(* Logix 5000 AddOnInstructionDefinition export Banner_Q90RKU_Param_v4; software revision 33.00 *)

TYPE Banner_IOL_Port_v4 :   // UDT that has all of the data items necessary to communicate with a specific Port on a IO-Link Master
STRUCT
   Port_Controlled : INT;   // Each bit represents a port on an IO-Link Master. Set to 1 to tell AOI to control that port.
   Port_Activate : INT;   // Each bit represents a port on an IO-Link Master. When ON that port will process any commands in queue.
   Port_Read : INT;   // Each bit represents a port on an IO-Link Master. Used to determine when device AOI has requested a Read command.
   Port_Write : INT;   // Each bit represents a port on an IO-Link Master. Used to determine when device AOI has requested a Write command.
   Port_RW_Complete : INT;   // Each bit represents a port on an IO-Link Master. Tells device AOI that Read or Write request has been completed.
   Port_Device_Read : INT;
   Data_Transfer : SINT[190];   // Array to transfer data from IO-Master to device AOIs.
END_STRUCT
END_TYPE

TYPE Banner_Q90RKU_Analog_v4 :
STRUCT
   AO1_SP1 : DINT;
   AO1_SP2 : DINT;
   AO1_Output_Type : INT;   // 0 = 4-20 mA, 128 = 0-10V, 129 = .5-4.5V
   AO1_Slope : SINT;   // 0 = Positive, 1 = Negative
   AO1_Loss_of_Signal : SINT;   // 0 = Hold, 1 = Low, 2 = High
   AO1_Average : SINT;   // 0 = 1, 1 = 2, 2= 4, 3 = 8, 4 = 16, 5 = 32, 6 = 64, 7 = 128, 8 = 256, 9 = 512
END_STRUCT
END_TYPE

TYPE Banner_Q90RKU_BDC_v4 :
STRUCT
   SP1 : DINT;   // Switchpoint SP1 switch point in Switch or Window mode.
   SP2 : DINT;   // Switchpoint 2. SP2 switch point in Window mode only.
   SP_Logic : INT;   // 0 = Light Operate, 1 = Dark Operate
   Mode : SINT;   // 1 = Switch Mode/Single Mode, 2 = Window Mode
   Hysteresis : INT;
   Delay_On : DINT;   // 0 to 60000 ms
   Delay_Off : DINT;   // 0 to 60000 ms
   Teach_Offset : DINT;   // Offset applied to taught switch point during single point teach.
END_STRUCT
END_TYPE

TYPE Banner_Q90RKU_Config_v4 :
STRUCT
   Response_Speed : SINT;   // 0 = Fast, 1 = Medium, 2 = Slow
   Peak_Select_Mode : SINT;   // 0 = Strongest Peak, 1 = First Peak
   Output_Polarity : SINT;   // 0 = NPN, 1 = PNP
   Process_Data_Filter_Time : INT;
   Process_Data_Layout : SINT;   // 0 = Digital Measurement Sensor, 1 = Distance and Excess Gain, 2 = Distance and Excess Gain with Binary Data
   Remote_Input_Mode : SINT;   // 0 = Disabled, 1 = Teach
   LEDs_Disabled : SINT;   // 0 = Enabled, 1 = Disabled.
   Amplitude_Threshold : DINT;   // 100 to 10000.
   Limit_Filter_Enabled : SINT;   // 0 = Disabled, 1 = Enabled. Rate of change filter for the distance measurement.
   Limit_Filter_Positive_Hold_Time : DINT;   // 50 to 3600000. Hold time for when distance change exceeds configured window.
   Limit_Filter_Negative_Hold_Time : DINT;   // 50 to 3600000. Hold time for when distance change exceeds configured window.
   Limit_Filter_Positive_Distance : DINT;   // 0 to 1000. Window size for distance changes going away from sensor (set to 0 to disable)
   Limit_Filter_Negative_Distance : DINT;   // 0 to 1000. Window size for distance changes goin towards sensor (set to 0 to disable)
END_STRUCT
END_TYPE

TYPE Banner_Q90RKU_Direct_v4 :
STRUCT
   Master_Cycle_Time : INT;
   Min_Cycle_Time : INT;
   M_Sequence_Capability : INT;
   IO_Link_Version_ID : INT;
   Process_Data_Input_Length : INT;
   Process_Data_Output_Length : INT;
   Combined_Vendor_ID : DINT;   // IO-Link Vendor ID
   Vendor_ID1 : INT;
   Vendor_ID2 : INT;
   Combined_Device_ID : DINT;   // IO-Link Device ID
   Device_ID1 : INT;
   Device_ID2 : INT;
   Device_ID3 : INT;
END_STRUCT
END_TYPE

TYPE Banner_Q90RKU_RD_v4 :   // UDT that stores the Read Data for a Q90RKU.
STRUCT
   Direct : Banner_Q90RKU_Direct_v4;
   Serial_Number : STRING;
   Teach_State : SINT;
   SP1_TP1 : SINT;
   SP1_TP2 : SINT;
   SP2_TP1 : SINT;
   SP2_TP2 : SINT;
   Status : Banner_Q90RKU_Status_v4;
   All_Time_Run_Time : DINT;   // Read only counter that tracks the total time sensor has been running since manufacture. Value in Hours.
   MDC_Lower_Limit : DINT;
   MDC_Upper_Limit : DINT;
   MDC_Unit : INT;
   MDC_Scale : SINT;
END_STRUCT
END_TYPE

TYPE Banner_Q90RKU_Status_v4 :
STRUCT
   Distance_Meaurement : DINT;
   Excess_Gain : DINT;   // Amount of singla measured over the minimum threshold.
   Stability : SINT;
   Fault_Status : SINT;   // 0 = No Fault, 1 = Fault Present
   Analog_Output_Value : DINT;
   Temperature : DINT;
   Last_Taught_Temperature : DINT;   // Internal Temperature the last time device was taught.
END_STRUCT
END_TYPE

TYPE Banner_Q90RKU_v4 :   // All of the parameters for a Q90RKU.
STRUCT
   Initial_Global_Read : BOOL;   // Determines if all of the IO-Link data has been read into the PLC yet
   Command : INT;   // Value placed in here will activate a read or write to a specifc IO-Link Index
   Read : Banner_Q90RKU_RD_v4;   // Read Only Data
   Write : Banner_Q90RKU_WD_v4;   // Write Data
   Archive : Banner_Q90RKU_WD_v4;   // Archive Data
   Reset : BOOL;   // Resets AOI. This will force a complete parameter read of the sensor.
END_STRUCT
END_TYPE

TYPE Banner_Q90RKU_WD_v4 :   // UDT that stores the Write Data for a T30RKU.
STRUCT
   System_Command : INT;   // See IODD file for list of commands that can be activated via the System Command interface
   Teach_in_Channel : SINT;   // 0 = Default, 1 = BDC1, 192 = AO1
   BDC1 : Banner_Q90RKU_BDC_v4;
   Config : Banner_Q90RKU_Config_v4;
   Resettable_Run_Time : DINT;
   All_Time_Run_Time_Event_Time : DINT;
   Resettable_Run_Time_Event_Time : DINT;
   Analog : Banner_Q90RKU_Analog_v4;
   Active_Sensing_Range_Near : DINT;
   Active_Sensing_Range_Far : DINT;
END_STRUCT
END_TYPE

ADD_ON_INSTRUCTION Banner_Q90RKU_Param_v4   (* revision 4.1, vendor Banner Engineering *)
// AOI to read and write parameter data to an IO-Link Q90R Analog.
VAR_IN_OUT
   Q90RKU : Banner_Q90RKU_v4; {required}
   Port_Data : Banner_IOL_Port_v4; {required}
END_VAR
VAR_INPUT
   Port : DINT; {required}
END_VAR
VAR
   Local_Control : DINT; {access None}
   Global_Read_Command_Value : INT; {access None}
   Global_Write_Command_Value : INT; {access None}
   Command_Being_Processed : BOOL; {access None}
   Update_Archive : BOOL; {access None}
   Index_Write_Inprocess : DINT; {access None}
   Index_Write_Control : DINT; {access None}
   Inprocess_Index : DINT; {access None}
END_VAR

ROUTINE Logic   (* ladder *)
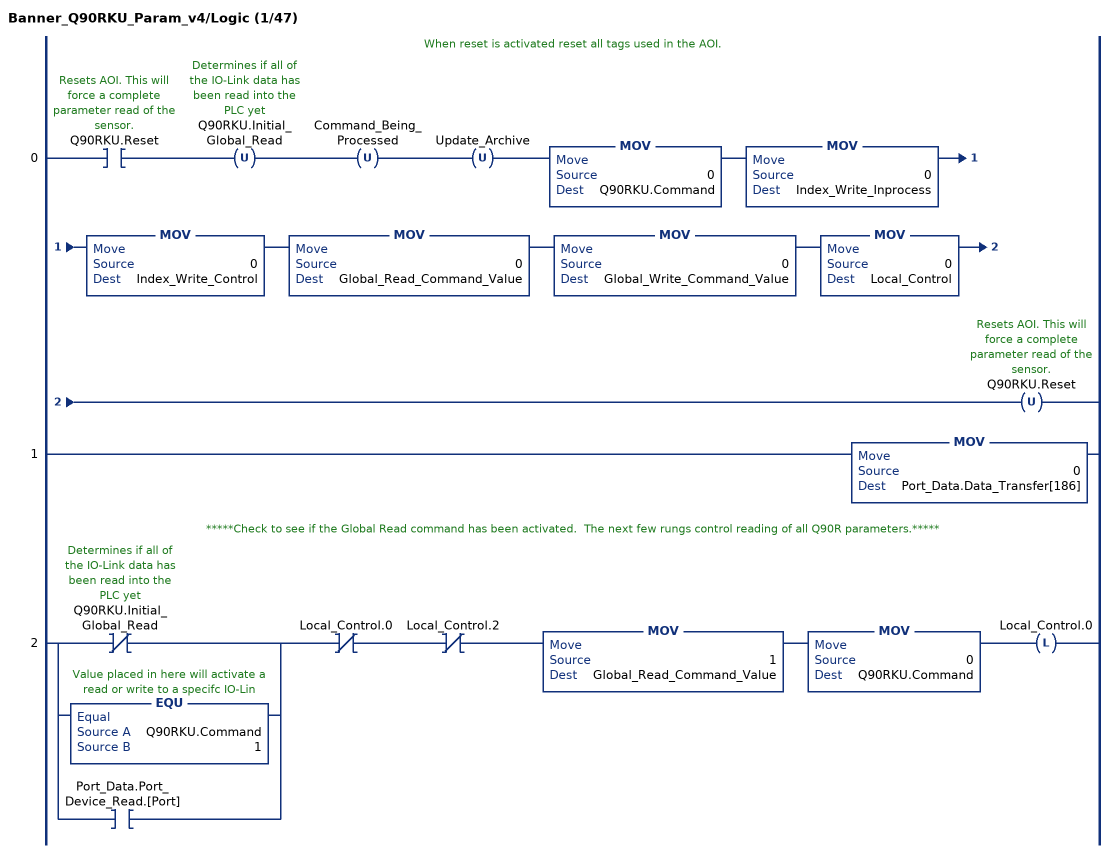
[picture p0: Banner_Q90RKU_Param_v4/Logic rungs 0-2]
   // When reset is activated reset all tags used in the AOI.
   0: XIC(Q90RKU.Reset)OTU(Q90RKU.Initial_Global_Read)OTU(Command_Being_Processed)OTU(Update_Archive)MOV(0,Q90RKU.Command)MOV(0,Index_Write_Inprocess)MOV(0,Index_Write_Control)MOV(0,Global_Read_Command_Value)MOV(0,Global_Write_Command_Value)MOV(0,Local_Control)OTU(Q90RKU.Reset);
   1: MOV(0,Port_Data.Data_Transfer[186]);
   // *****Check to see if the Global Read command has been activated.  The next few rungs control reading of all Q90R parameters.*****
   2: [XIO(Q90RKU.Initial_Global_Read) ,EQU(Q90RKU.Command,1) ,XIC(Port_Data.Port_Device_Read.[Port]) ]XIO(Local_Control.0)XIO(Local_Control.2)MOV(1,Global_Read_Command_Value)MOV(0,Q90RKU.Command)OTL(Local_Control.0);
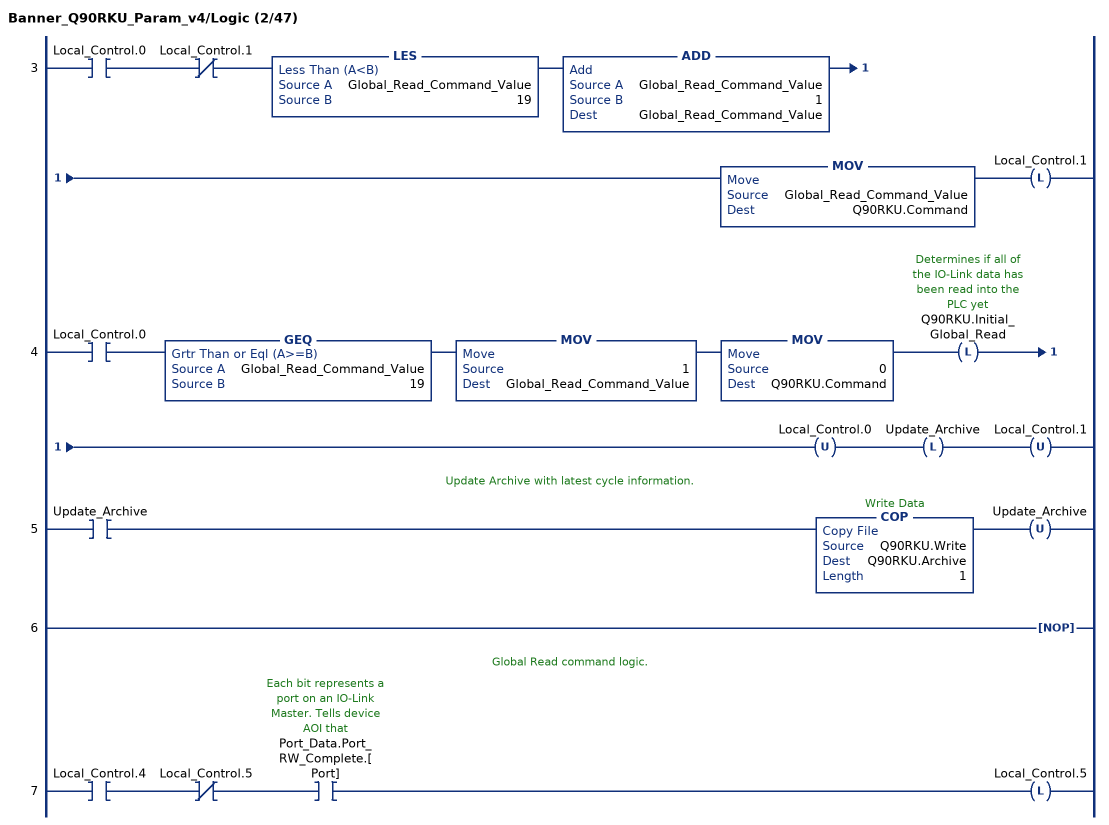
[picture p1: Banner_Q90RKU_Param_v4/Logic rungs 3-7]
   3: XIC(Local_Control.0)XIO(Local_Control.1)LES(Global_Read_Command_Value,19)ADD(Global_Read_Command_Value,1,Global_Read_Command_Value)MOV(Global_Read_Command_Value,Q90RKU.Command)OTL(Local_Control.1);
   4: XIC(Local_Control.0)GEQ(Global_Read_Command_Value,19)MOV(1,Global_Read_Command_Value)MOV(0,Q90RKU.Command)OTL(Q90RKU.Initial_Global_Read)OTU(Local_Control.0)OTL(Update_Archive)OTU(Local_Control.1);
   // Update Archive with latest cycle information.
   5: XIC(Update_Archive)COP(Q90RKU.Write,Q90RKU.Archive,1)OTU(Update_Archive);
   6: NOP();
   // Global Read command logic.
   7: XIC(Local_Control.4)XIO(Local_Control.5)XIC(Port_Data.Port_RW_Complete.[Port])OTL(Local_Control.5);
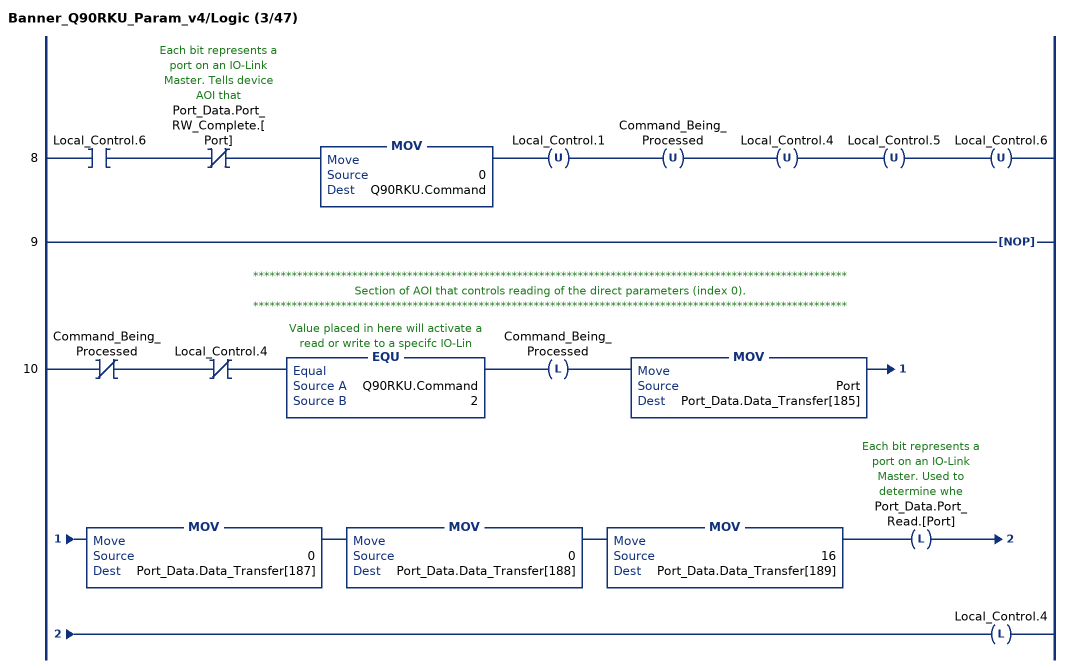
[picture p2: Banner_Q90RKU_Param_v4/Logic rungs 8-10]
   8: XIC(Local_Control.6)XIO(Port_Data.Port_RW_Complete.[Port])MOV(0,Q90RKU.Command)OTU(Local_Control.1)OTU(Command_Being_Processed)OTU(Local_Control.4)OTU(Local_Control.5)OTU(Local_Control.6);
   9: NOP();
   // ************************************************************************************************************
   // Section of AOI that controls reading of the direct parameters (index 0).
   // ************************************************************************************************************
   10: XIO(Command_Being_Processed)XIO(Local_Control.4)EQU(Q90RKU.Command,2)OTL(Command_Being_Processed)MOV(Port,Port_Data.Data_Transfer[185])MOV(0,Port_Data.Data_Transfer[187])MOV(0,Port_Data.Data_Transfer[188])MOV(16,Port_Data.Data_Transfer[189])OTL(Port_Data.Port_Read.[Port])OTL(Local_Control.4);
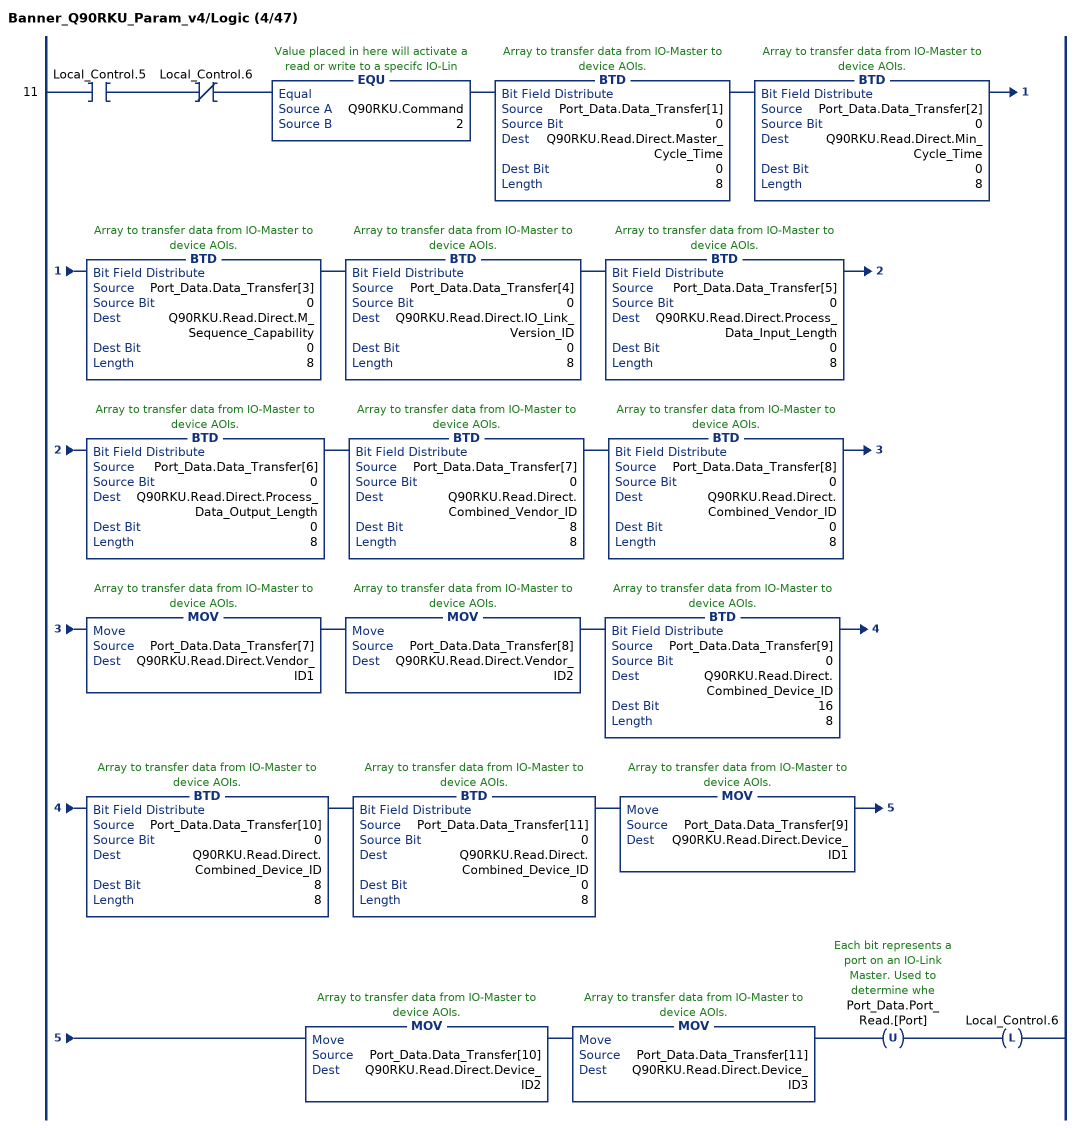
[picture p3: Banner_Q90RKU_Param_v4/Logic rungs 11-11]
   11: XIC(Local_Control.5)XIO(Local_Control.6)EQU(Q90RKU.Command,2)BTD(Port_Data.Data_Transfer[1],0,Q90RKU.Read.Direct.Master_Cycle_Time,0,8)BTD(Port_Data.Data_Transfer[2],0,Q90RKU.Read.Direct.Min_Cycle_Time,0,8)BTD(Port_Data.Data_Transfer[3],0,Q90RKU.Read.Direct.M_Sequence_Capability,0,8)BTD(Port_Data.Data_Transfer[4],0,Q90RKU.Read.Direct.IO_Link_Version_ID,0,8)BTD(Port_Data.Data_Transfer[5],0,Q90RKU.Read.Direct.Process_Data_Input_Length,0,8)BTD(Port_Data.Data_Transfer[6],0,Q90RKU.Read.Direct.Process_Data_Output_Length,0,8)BTD(Port_Data.Data_Transfer[7],0,Q90RKU.Read.Direct.Combined_Vendor_ID,8,8)BTD(Port_Data.Data_Transfer[8],0,Q90RKU.Read.Direct.Combined_Vendor_ID,0,8)MOV(Port_Data.Data_Transfer[7],Q90RKU.Read.Direct.Vendor_ID1)MOV(Port_Data.Data_Transfer[8],Q90RKU.Read.Direct.Vendor_ID2)BTD(Port_Data.Data_Transfer[9],0,Q90RKU.Read.Direct.Combined_Device_ID,16,8)BTD(Port_Data.Data_Transfer[10],0,Q90RKU.Read.Direct.Combined_Device_ID,8,8)BTD(Port_Data.Data_Transfer[11],0,Q90RKU.Read.Direct.Combined_Device_ID,0,8)MOV(Port_Data.Data_Transfer[9],Q90RKU.Read.Direct.Device_ID1)MOV(Port_Data.Data_Transfer[10],Q90RKU.Read.Direct.Device_ID2)MOV(Port_Data.Data_Transfer[11],Q90RKU.Read.Direct.Device_ID3)OTU(Port_Data.Port_Read.[Port])OTL(Local_Control.6);
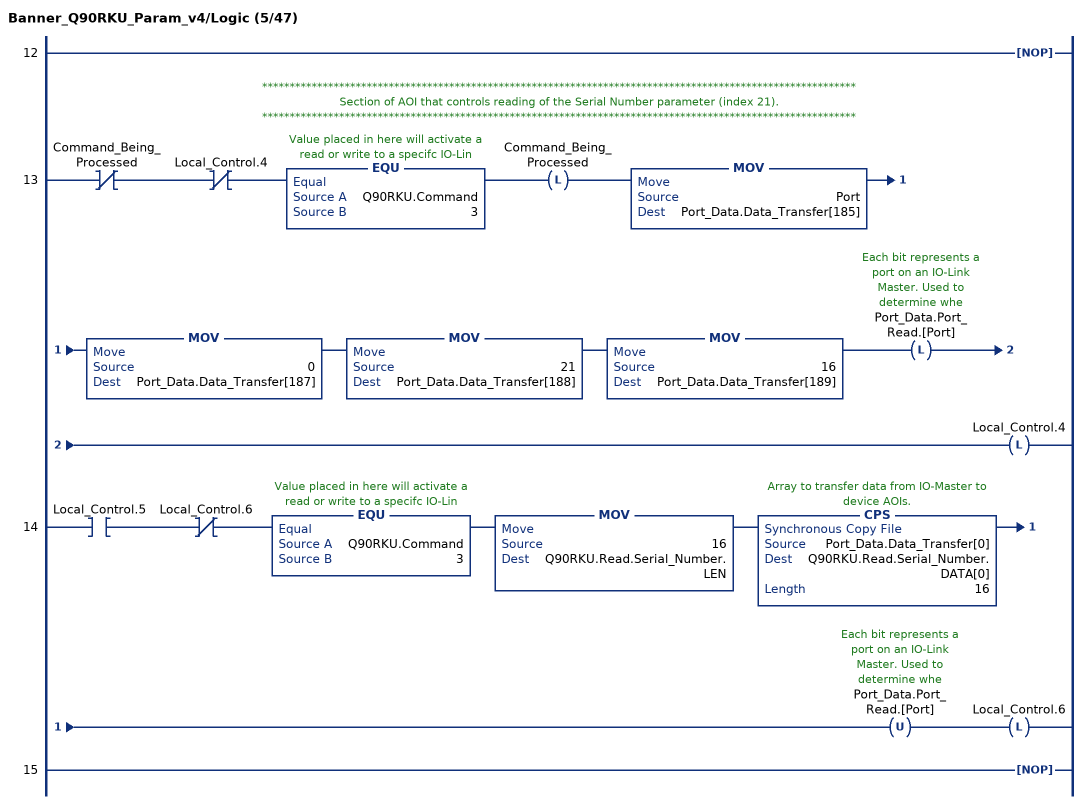
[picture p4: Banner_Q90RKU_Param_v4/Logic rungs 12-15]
   12: NOP();
   // ************************************************************************************************************
   // Section of AOI that controls reading of the Serial Number parameter (index 21).
   // ************************************************************************************************************
   13: XIO(Command_Being_Processed)XIO(Local_Control.4)EQU(Q90RKU.Command,3)OTL(Command_Being_Processed)MOV(Port,Port_Data.Data_Transfer[185])MOV(0,Port_Data.Data_Transfer[187])MOV(21,Port_Data.Data_Transfer[188])MOV(16,Port_Data.Data_Transfer[189])OTL(Port_Data.Port_Read.[Port])OTL(Local_Control.4);
   14: XIC(Local_Control.5)XIO(Local_Control.6)EQU(Q90RKU.Command,3)MOV(16,Q90RKU.Read.Serial_Number.LEN)CPS(Port_Data.Data_Transfer[0],Q90RKU.Read.Serial_Number.DATA[0],16)OTU(Port_Data.Port_Read.[Port])OTL(Local_Control.6);
   15: NOP();
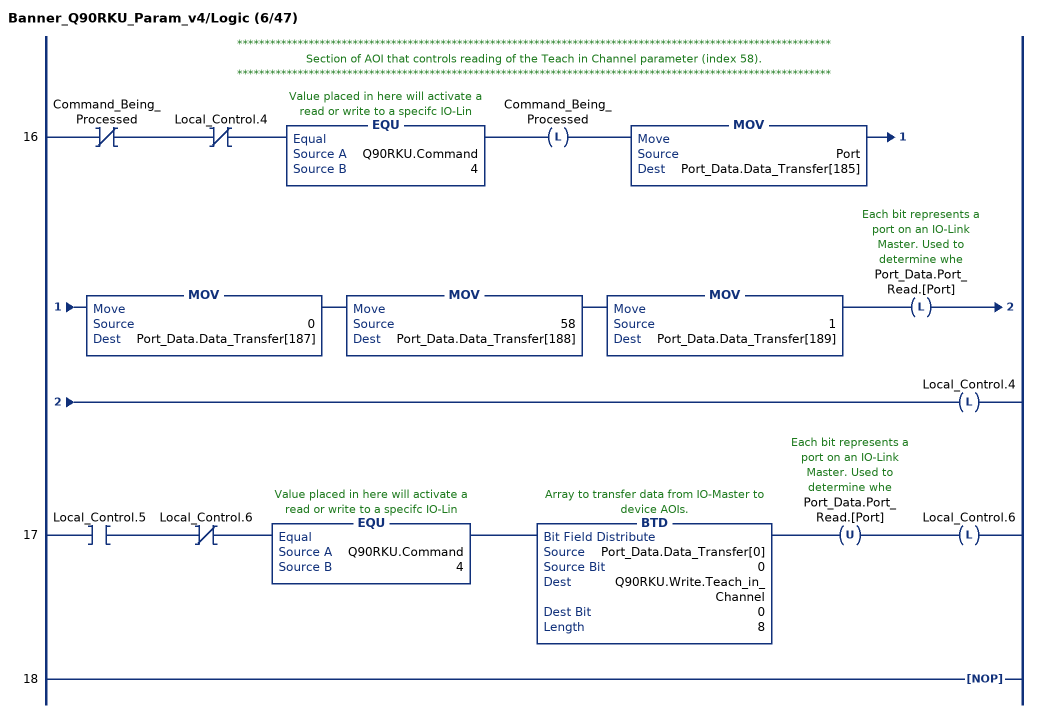
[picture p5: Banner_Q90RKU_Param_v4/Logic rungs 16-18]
   // ************************************************************************************************************
   // Section of AOI that controls reading of the Teach in Channel parameter (index 58).
   // ************************************************************************************************************
   16: XIO(Command_Being_Processed)XIO(Local_Control.4)EQU(Q90RKU.Command,4)OTL(Command_Being_Processed)MOV(Port,Port_Data.Data_Transfer[185])MOV(0,Port_Data.Data_Transfer[187])MOV(58,Port_Data.Data_Transfer[188])MOV(1,Port_Data.Data_Transfer[189])OTL(Port_Data.Port_Read.[Port])OTL(Local_Control.4);
   17: XIC(Local_Control.5)XIO(Local_Control.6)EQU(Q90RKU.Command,4)BTD(Port_Data.Data_Transfer[0],0,Q90RKU.Write.Teach_in_Channel,0,8)OTU(Port_Data.Port_Read.[Port])OTL(Local_Control.6);
   18: NOP();
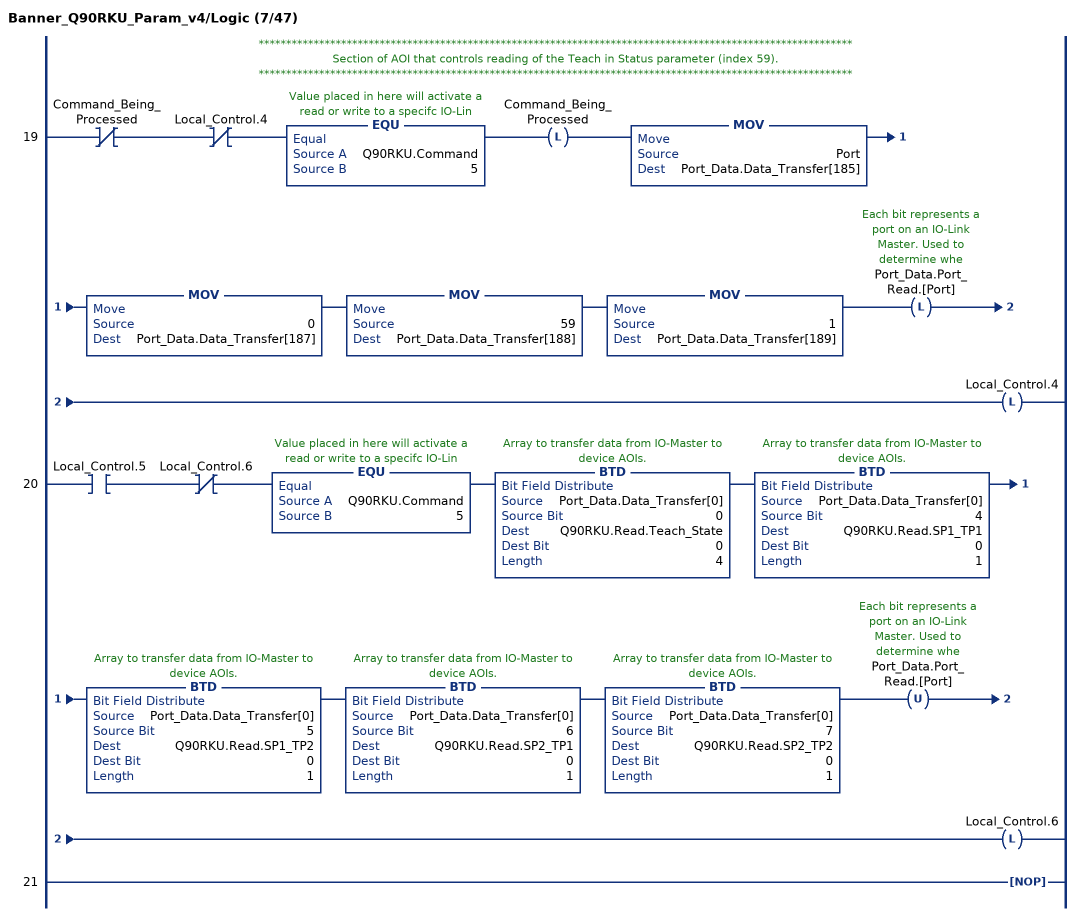
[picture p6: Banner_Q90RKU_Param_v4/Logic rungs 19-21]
   // ************************************************************************************************************
   // Section of AOI that controls reading of the Teach in Status parameter (index 59).
   // ************************************************************************************************************
   19: XIO(Command_Being_Processed)XIO(Local_Control.4)EQU(Q90RKU.Command,5)OTL(Command_Being_Processed)MOV(Port,Port_Data.Data_Transfer[185])MOV(0,Port_Data.Data_Transfer[187])MOV(59,Port_Data.Data_Transfer[188])MOV(1,Port_Data.Data_Transfer[189])OTL(Port_Data.Port_Read.[Port])OTL(Local_Control.4);
   20: XIC(Local_Control.5)XIO(Local_Control.6)EQU(Q90RKU.Command,5)BTD(Port_Data.Data_Transfer[0],0,Q90RKU.Read.Teach_State,0,4)BTD(Port_Data.Data_Transfer[0],4,Q90RKU.Read.SP1_TP1,0,1)BTD(Port_Data.Data_Transfer[0],5,Q90RKU.Read.SP1_TP2,0,1)BTD(Port_Data.Data_Transfer[0],6,Q90RKU.Read.SP2_TP1,0,1)BTD(Port_Data.Data_Transfer[0],7,Q90RKU.Read.SP2_TP2,0,1)OTU(Port_Data.Port_Read.[Port])OTL(Local_Control.6);
   21: NOP();
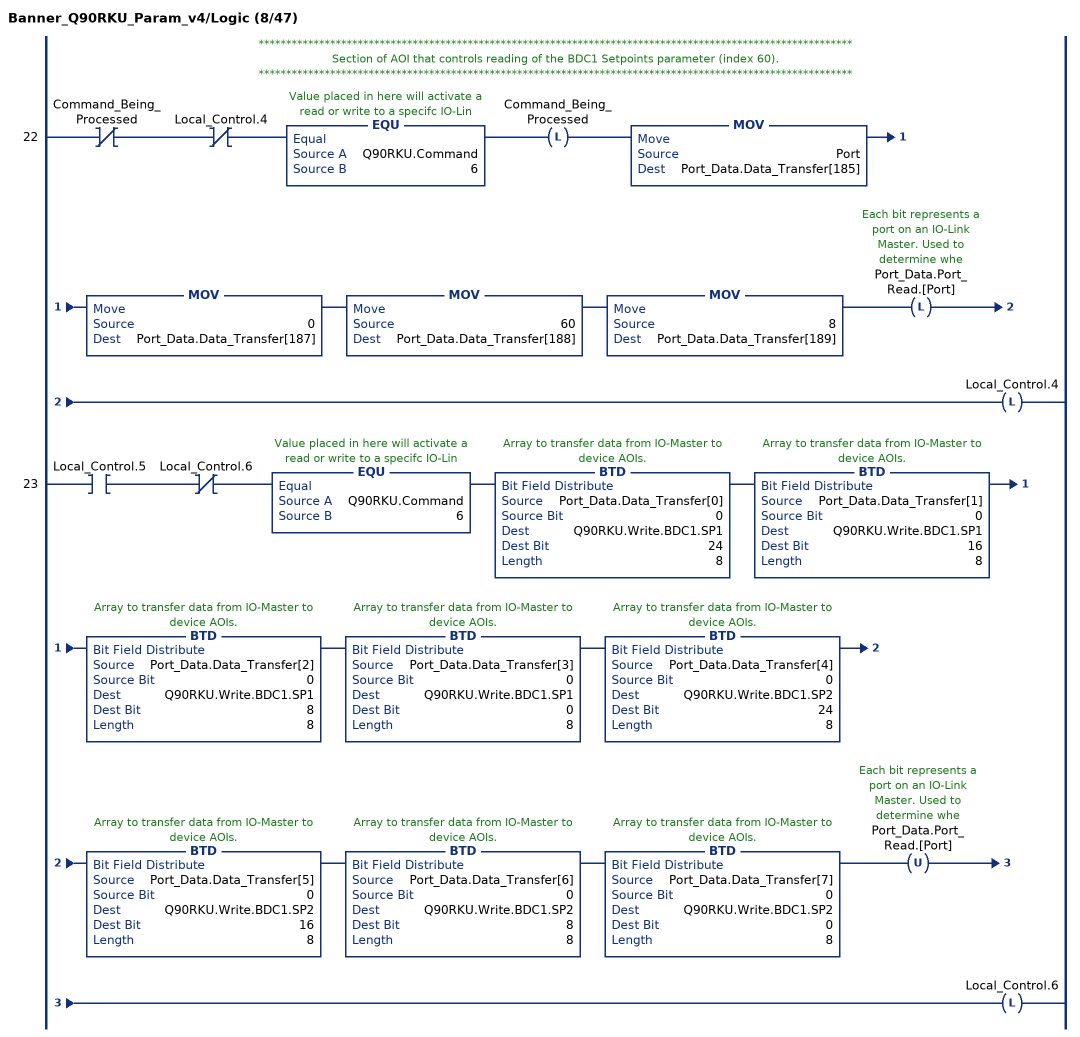
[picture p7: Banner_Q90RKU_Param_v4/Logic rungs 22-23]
   // ************************************************************************************************************
   // Section of AOI that controls reading of the BDC1 Setpoints parameter (index 60).
   // ************************************************************************************************************
   22: XIO(Command_Being_Processed)XIO(Local_Control.4)EQU(Q90RKU.Command,6)OTL(Command_Being_Processed)MOV(Port,Port_Data.Data_Transfer[185])MOV(0,Port_Data.Data_Transfer[187])MOV(60,Port_Data.Data_Transfer[188])MOV(8,Port_Data.Data_Transfer[189])OTL(Port_Data.Port_Read.[Port])OTL(Local_Control.4);
   23: XIC(Local_Control.5)XIO(Local_Control.6)EQU(Q90RKU.Command,6)BTD(Port_Data.Data_Transfer[0],0,Q90RKU.Write.BDC1.SP1,24,8)BTD(Port_Data.Data_Transfer[1],0,Q90RKU.Write.BDC1.SP1,16,8)BTD(Port_Data.Data_Transfer[2],0,Q90RKU.Write.BDC1.SP1,8,8)BTD(Port_Data.Data_Transfer[3],0,Q90RKU.Write.BDC1.SP1,0,8)BTD(Port_Data.Data_Transfer[4],0,Q90RKU.Write.BDC1.SP2,24,8)BTD(Port_Data.Data_Transfer[5],0,Q90RKU.Write.BDC1.SP2,16,8)BTD(Port_Data.Data_Transfer[6],0,Q90RKU.Write.BDC1.SP2,8,8)BTD(Port_Data.Data_Transfer[7],0,Q90RKU.Write.BDC1.SP2,0,8)OTU(Port_Data.Port_Read.[Port])OTL(Local_Control.6);
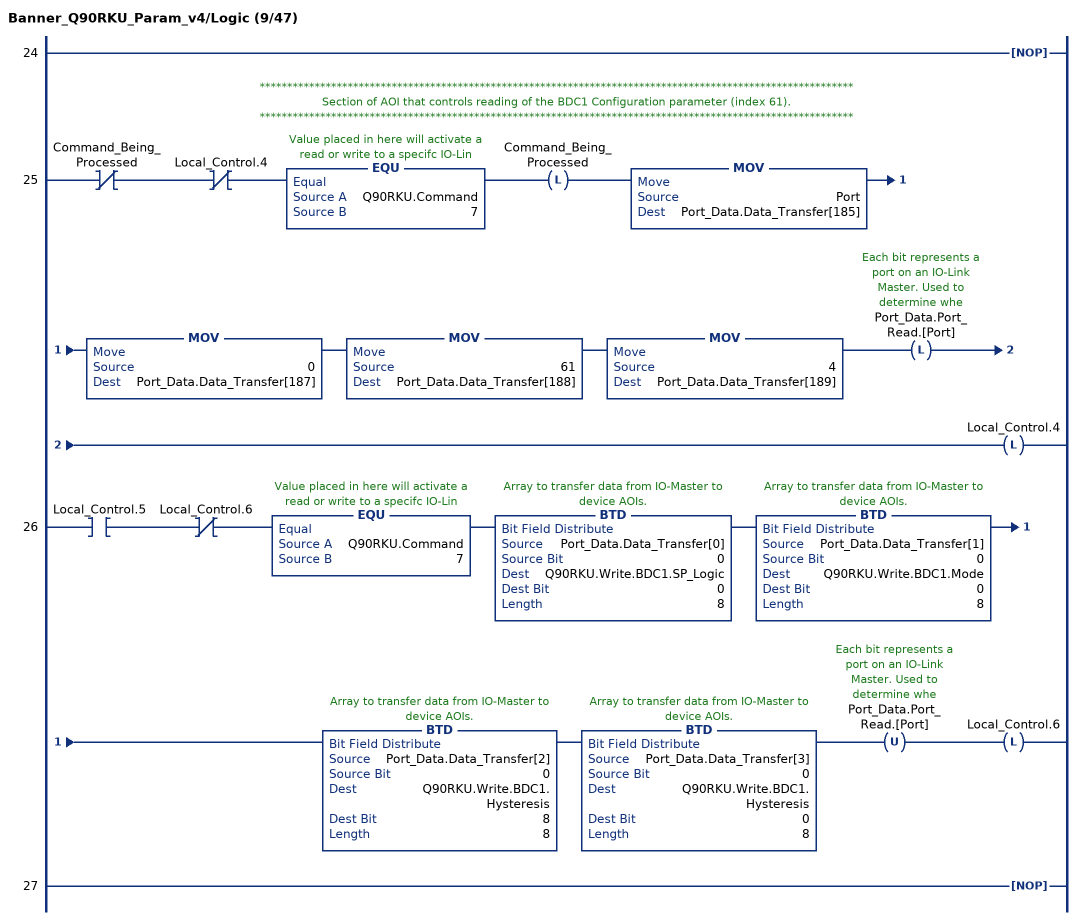
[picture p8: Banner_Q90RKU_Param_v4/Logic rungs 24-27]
   24: NOP();
   // ************************************************************************************************************
   // Section of AOI that controls reading of the BDC1 Configuration parameter (index 61).
   // ************************************************************************************************************
   25: XIO(Command_Being_Processed)XIO(Local_Control.4)EQU(Q90RKU.Command,7)OTL(Command_Being_Processed)MOV(Port,Port_Data.Data_Transfer[185])MOV(0,Port_Data.Data_Transfer[187])MOV(61,Port_Data.Data_Transfer[188])MOV(4,Port_Data.Data_Transfer[189])OTL(Port_Data.Port_Read.[Port])OTL(Local_Control.4);
   26: XIC(Local_Control.5)XIO(Local_Control.6)EQU(Q90RKU.Command,7)BTD(Port_Data.Data_Transfer[0],0,Q90RKU.Write.BDC1.SP_Logic,0,8)BTD(Port_Data.Data_Transfer[1],0,Q90RKU.Write.BDC1.Mode,0,8)BTD(Port_Data.Data_Transfer[2],0,Q90RKU.Write.BDC1.Hysteresis,8,8)BTD(Port_Data.Data_Transfer[3],0,Q90RKU.Write.BDC1.Hysteresis,0,8)OTU(Port_Data.Port_Read.[Port])OTL(Local_Control.6);
   27: NOP();
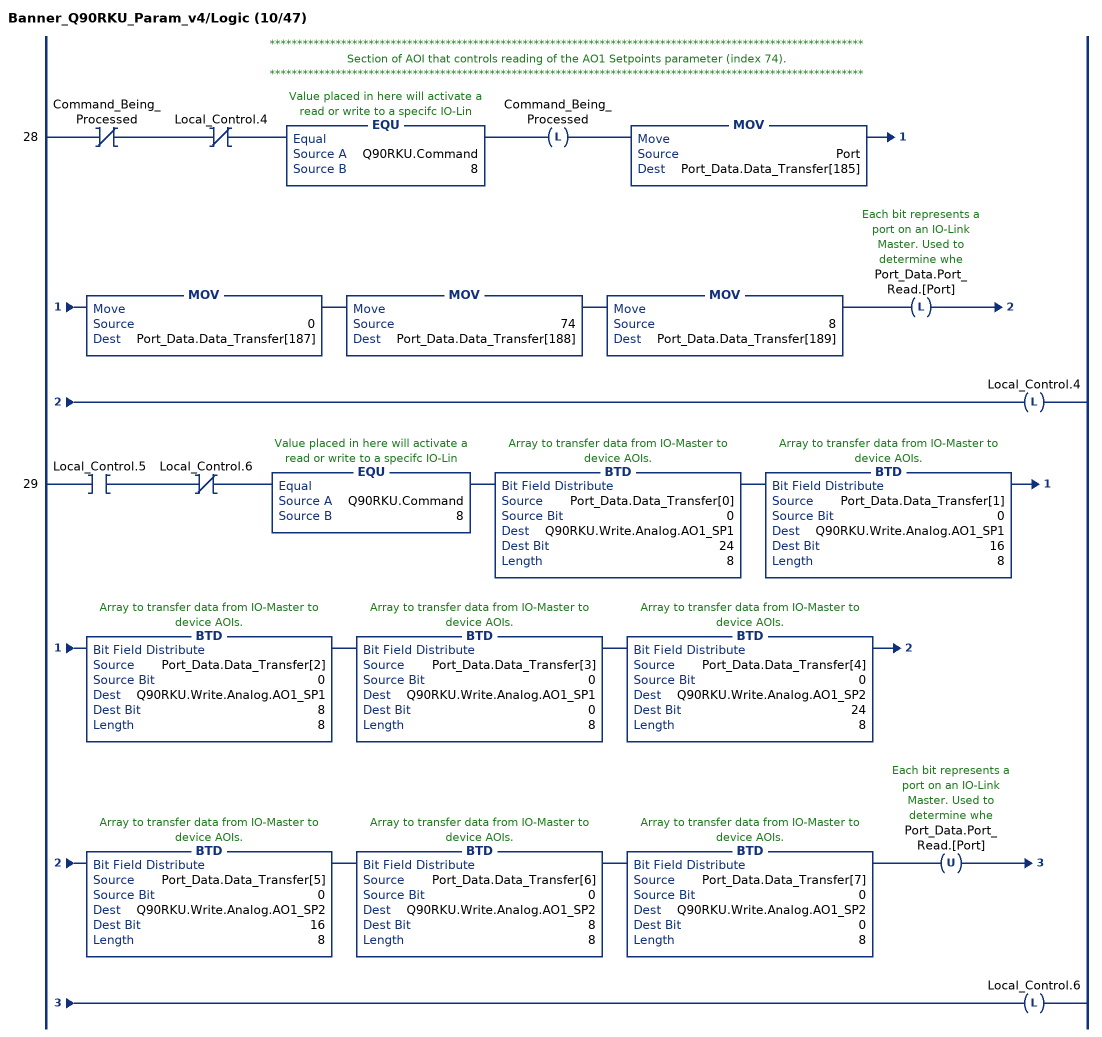
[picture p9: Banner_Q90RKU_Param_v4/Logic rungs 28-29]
   // ************************************************************************************************************
   // Section of AOI that controls reading of the AO1 Setpoints parameter (index 74).
   // ************************************************************************************************************
   28: XIO(Command_Being_Processed)XIO(Local_Control.4)EQU(Q90RKU.Command,8)OTL(Command_Being_Processed)MOV(Port,Port_Data.Data_Transfer[185])MOV(0,Port_Data.Data_Transfer[187])MOV(74,Port_Data.Data_Transfer[188])MOV(8,Port_Data.Data_Transfer[189])OTL(Port_Data.Port_Read.[Port])OTL(Local_Control.4);
   29: XIC(Local_Control.5)XIO(Local_Control.6)EQU(Q90RKU.Command,8)BTD(Port_Data.Data_Transfer[0],0,Q90RKU.Write.Analog.AO1_SP1,24,8)BTD(Port_Data.Data_Transfer[1],0,Q90RKU.Write.Analog.AO1_SP1,16,8)BTD(Port_Data.Data_Transfer[2],0,Q90RKU.Write.Analog.AO1_SP1,8,8)BTD(Port_Data.Data_Transfer[3],0,Q90RKU.Write.Analog.AO1_SP1,0,8)BTD(Port_Data.Data_Transfer[4],0,Q90RKU.Write.Analog.AO1_SP2,24,8)BTD(Port_Data.Data_Transfer[5],0,Q90RKU.Write.Analog.AO1_SP2,16,8)BTD(Port_Data.Data_Transfer[6],0,Q90RKU.Write.Analog.AO1_SP2,8,8)BTD(Port_Data.Data_Transfer[7],0,Q90RKU.Write.Analog.AO1_SP2,0,8)OTU(Port_Data.Port_Read.[Port])OTL(Local_Control.6);
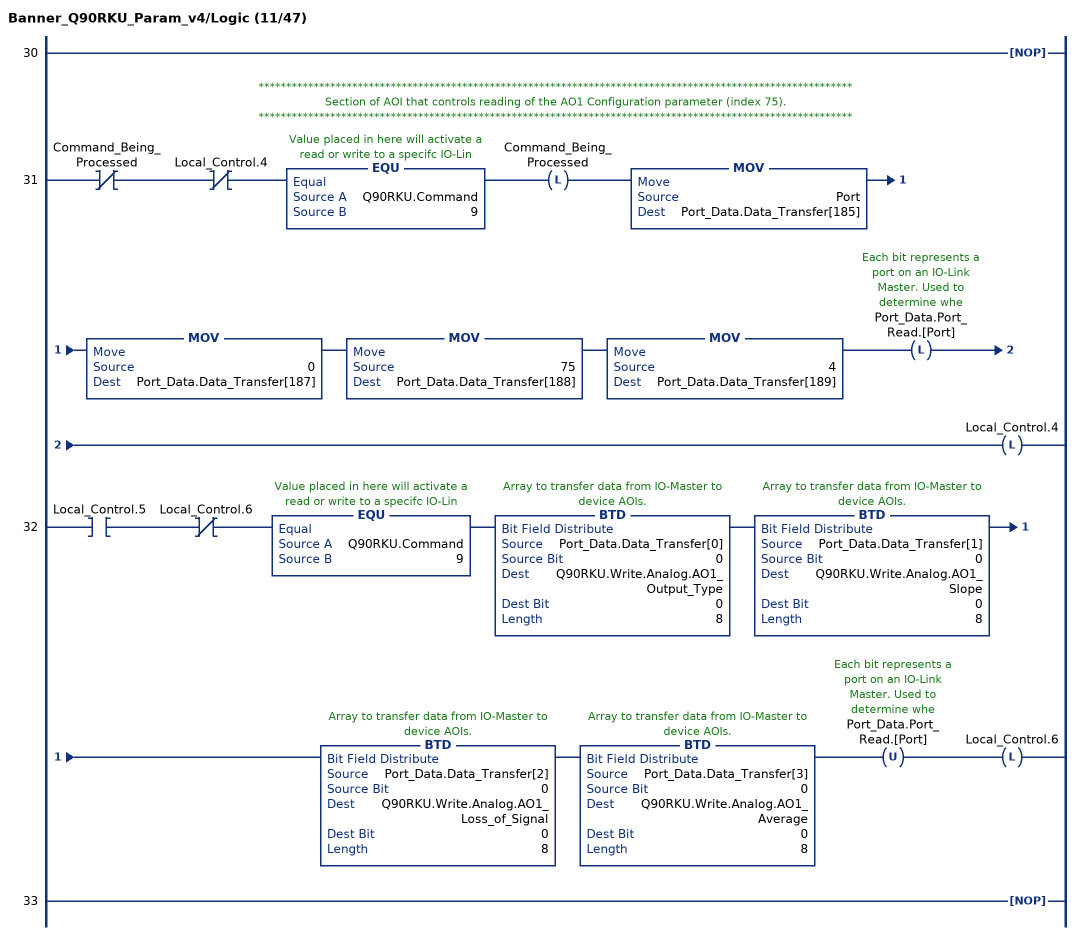
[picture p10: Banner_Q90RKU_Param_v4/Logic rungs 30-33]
   30: NOP();
   // ************************************************************************************************************
   // Section of AOI that controls reading of the AO1 Configuration parameter (index 75).
   // ************************************************************************************************************
   31: XIO(Command_Being_Processed)XIO(Local_Control.4)EQU(Q90RKU.Command,9)OTL(Command_Being_Processed)MOV(Port,Port_Data.Data_Transfer[185])MOV(0,Port_Data.Data_Transfer[187])MOV(75,Port_Data.Data_Transfer[188])MOV(4,Port_Data.Data_Transfer[189])OTL(Port_Data.Port_Read.[Port])OTL(Local_Control.4);
   32: XIC(Local_Control.5)XIO(Local_Control.6)EQU(Q90RKU.Command,9)BTD(Port_Data.Data_Transfer[0],0,Q90RKU.Write.Analog.AO1_Output_Type,0,8)BTD(Port_Data.Data_Transfer[1],0,Q90RKU.Write.Analog.AO1_Slope,0,8)BTD(Port_Data.Data_Transfer[2],0,Q90RKU.Write.Analog.AO1_Loss_of_Signal,0,8)BTD(Port_Data.Data_Transfer[3],0,Q90RKU.Write.Analog.AO1_Average,0,8)OTU(Port_Data.Port_Read.[Port])OTL(Local_Control.6);
   33: NOP();
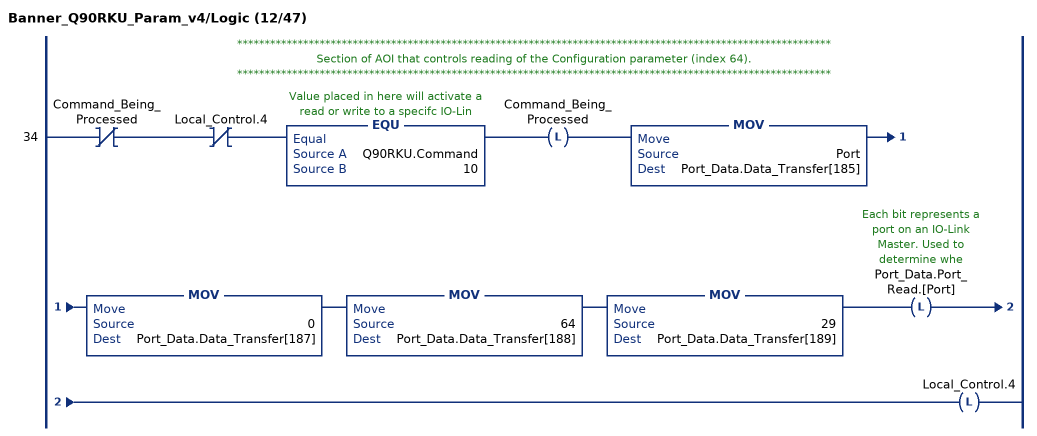
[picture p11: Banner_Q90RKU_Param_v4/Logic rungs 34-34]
   // ************************************************************************************************************
   // Section of AOI that controls reading of the Configuration parameter (index 64).
   // ************************************************************************************************************
   34: XIO(Command_Being_Processed)XIO(Local_Control.4)EQU(Q90RKU.Command,10)OTL(Command_Being_Processed)MOV(Port,Port_Data.Data_Transfer[185])MOV(0,Port_Data.Data_Transfer[187])MOV(64,Port_Data.Data_Transfer[188])MOV(29,Port_Data.Data_Transfer[189])OTL(Port_Data.Port_Read.[Port])OTL(Local_Control.4);
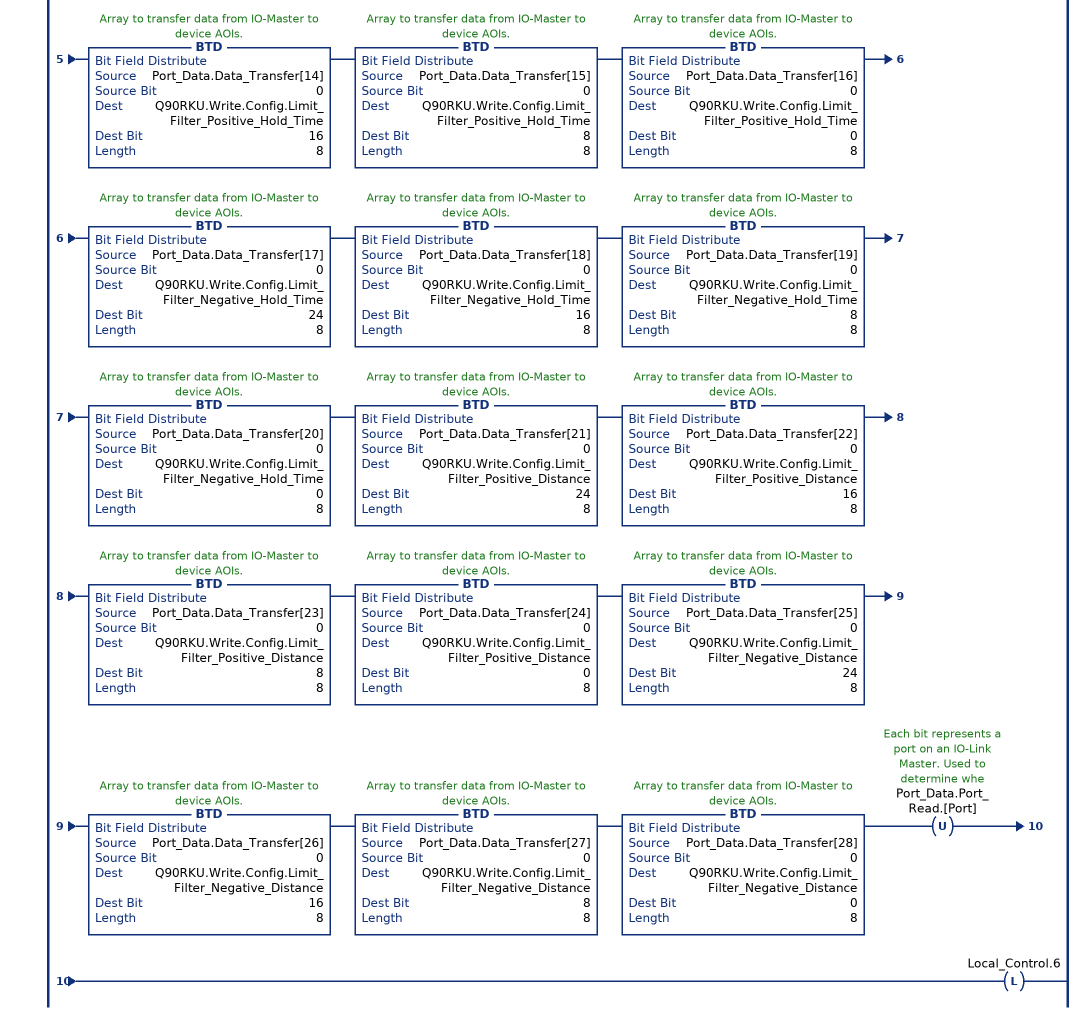
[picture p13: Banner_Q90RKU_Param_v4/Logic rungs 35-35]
   35: XIC(Local_Control.5)XIO(Local_Control.6)EQU(Q90RKU.Command,10)BTD(Port_Data.Data_Transfer[0],0,Q90RKU.Write.Config.Response_Speed,0,8)BTD(Port_Data.Data_Transfer[1],0,Q90RKU.Write.Config.Peak_Select_Mode,0,8)BTD(Port_Data.Data_Transfer[2],0,Q90RKU.Write.Config.Output_Polarity,0,8)BTD(Port_Data.Data_Transfer[3],0,Q90RKU.Write.Config.Process_Data_Filter_Time,8,8)BTD(Port_Data.Data_Transfer[4],0,Q90RKU.Write.Config.Process_Data_Filter_Time,0,8)BTD(Port_Data.Data_Transfer[5],0,Q90RKU.Write.Config.Process_Data_Layout,0,8)BTD(Port_Data.Data_Transfer[6],0,Q90RKU.Write.Config.Remote_Input_Mode,0,8)BTD(Port_Data.Data_Transfer[7],0,Q90RKU.Write.Config.LEDs_Disabled,0,8)BTD(Port_Data.Data_Transfer[8],0,Q90RKU.Write.Config.Amplitude_Threshold,24,8)BTD(Port_Data.Data_Transfer[9],0,Q90RKU.Write.Config.Amplitude_Threshold,16,8)BTD(Port_Data.Data_Transfer[10],0,Q90RKU.Write.Config.Amplitude_Threshold,8,8)BTD(Port_Data.Data_Transfer[11],0,Q90RKU.Write.Config.Amplitude_Threshold,0,8)BTD(Port_Data.Data_Transfer[12],0,Q90RKU.Write.Config.Limit_Filter_Enabled,0,8)BTD(Port_Data.Data_Transfer[13],0,Q90RKU.Write.Config.Limit_Filter_Positive_Hold_Time,24,8)BTD(Port_Data.Data_Transfer[14],0,Q90RKU.Write.Config.Limit_Filter_Positive_Hold_Time,16,8)BTD(Port_Data.Data_Transfer[15],0,Q90RKU.Write.Config.Limit_Filter_Positive_Hold_Time,8,8)BTD(Port_Data.Data_Transfer[16],0,Q90RKU.Write.Config.Limit_Filter_Positive_Hold_Time,0,8)BTD(Port_Data.Data_Transfer[17],0,Q90RKU.Write.Config.Limit_Filter_Negative_Hold_Time,24,8)BTD(Port_Data.Data_Transfer[18],0,Q90RKU.Write.Config.Limit_Filter_Negative_Hold_Time,16,8)BTD(Port_Data.Data_Transfer[19],0,Q90RKU.Write.Config.Limit_Filter_Negative_Hold_Time,8,8)BTD(Port_Data.Data_Transfer[20],0,Q90RKU.Write.Config.Limit_Filter_Negative_Hold_Time,0,8)BTD(Port_Data.Data_Transfer[21],0,Q90RKU.Write.Config.Limit_Filter_Positive_Distance,24,8)BTD(Port_Data.Data_Transfer[22],0,Q90RKU.Write.Config.Limit_Filter_Positive_Distance,16,8)BTD(Port_Data.Data_Transfer[23],0,Q90RKU.Write.Config.Limit_Filter_Positive_Distance,8,8)BTD(Port_Data.Data_Transfer[24],0,Q90RKU.Write.Config.Limit_Filter_Positive_Distance,0,8)BTD(Port_Data.Data_Transfer[25],0,Q90RKU.Write.Config.Limit_Filter_Negative_Distance,24,8)BTD(Port_Data.Data_Transfer[26],0,Q90RKU.Write.Config.Limit_Filter_Negative_Distance,16,8)BTD(Port_Data.Data_Transfer[27],0,Q90RKU.Write.Config.Limit_Filter_Negative_Distance,8,8)BTD(Port_Data.Data_Transfer[28],0,Q90RKU.Write.Config.Limit_Filter_Negative_Distance,0,8)OTU(Port_Data.Port_Read.[Port])OTL(Local_Control.6);
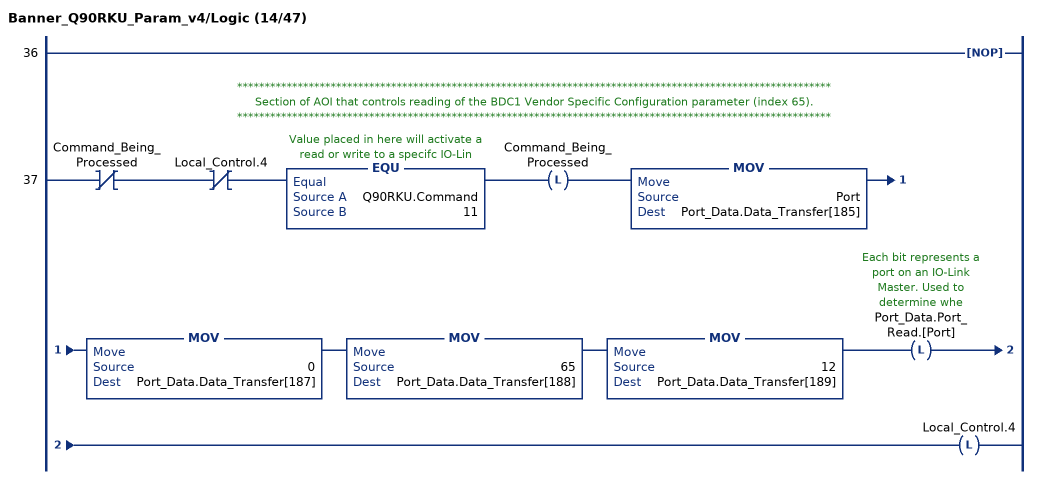
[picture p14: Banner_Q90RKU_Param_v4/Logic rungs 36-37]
   36: NOP();
   // ************************************************************************************************************
   // Section of AOI that controls reading of the BDC1 Vendor Specific Configuration parameter (index 65).
   // ************************************************************************************************************
   37: XIO(Command_Being_Processed)XIO(Local_Control.4)EQU(Q90RKU.Command,11)OTL(Command_Being_Processed)MOV(Port,Port_Data.Data_Transfer[185])MOV(0,Port_Data.Data_Transfer[187])MOV(65,Port_Data.Data_Transfer[188])MOV(12,Port_Data.Data_Transfer[189])OTL(Port_Data.Port_Read.[Port])OTL(Local_Control.4);
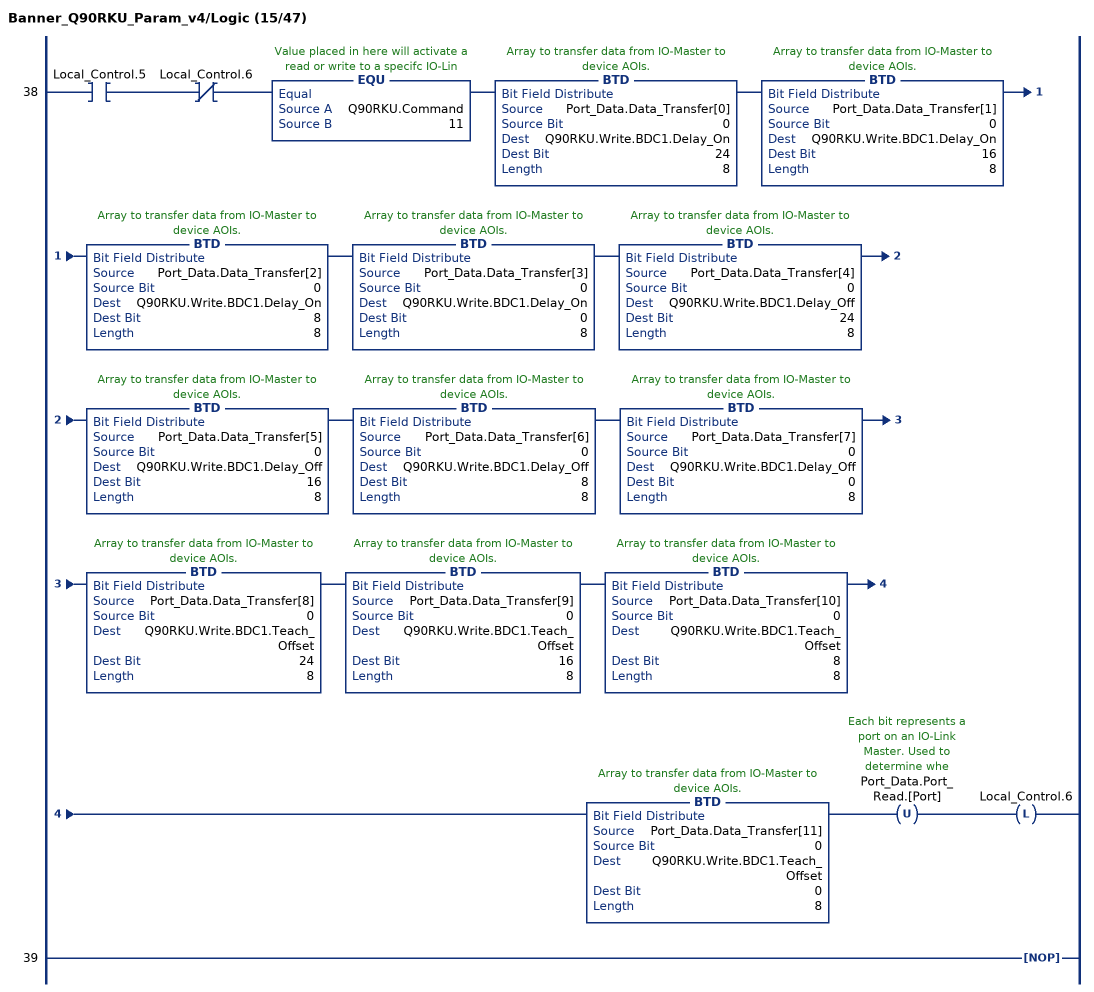
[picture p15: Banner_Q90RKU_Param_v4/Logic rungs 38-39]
   38: XIC(Local_Control.5)XIO(Local_Control.6)EQU(Q90RKU.Command,11)BTD(Port_Data.Data_Transfer[0],0,Q90RKU.Write.BDC1.Delay_On,24,8)BTD(Port_Data.Data_Transfer[1],0,Q90RKU.Write.BDC1.Delay_On,16,8)BTD(Port_Data.Data_Transfer[2],0,Q90RKU.Write.BDC1.Delay_On,8,8)BTD(Port_Data.Data_Transfer[3],0,Q90RKU.Write.BDC1.Delay_On,0,8)BTD(Port_Data.Data_Transfer[4],0,Q90RKU.Write.BDC1.Delay_Off,24,8)BTD(Port_Data.Data_Transfer[5],0,Q90RKU.Write.BDC1.Delay_Off,16,8)BTD(Port_Data.Data_Transfer[6],0,Q90RKU.Write.BDC1.Delay_Off,8,8)BTD(Port_Data.Data_Transfer[7],0,Q90RKU.Write.BDC1.Delay_Off,0,8)BTD(Port_Data.Data_Transfer[8],0,Q90RKU.Write.BDC1.Teach_Offset,24,8)BTD(Port_Data.Data_Transfer[9],0,Q90RKU.Write.BDC1.Teach_Offset,16,8)BTD(Port_Data.Data_Transfer[10],0,Q90RKU.Write.BDC1.Teach_Offset,8,8)BTD(Port_Data.Data_Transfer[11],0,Q90RKU.Write.BDC1.Teach_Offset,0,8)OTU(Port_Data.Port_Read.[Port])OTL(Local_Control.6);
   39: NOP();
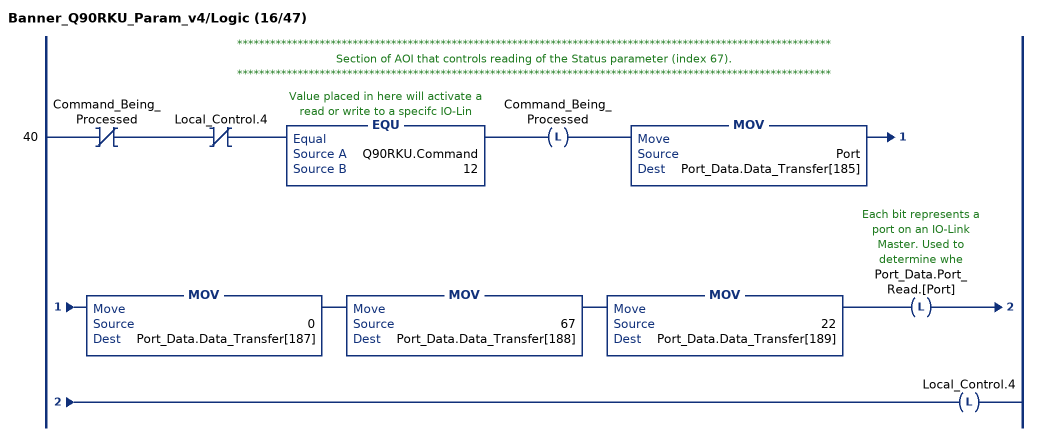
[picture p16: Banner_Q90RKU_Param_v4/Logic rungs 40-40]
   // ************************************************************************************************************
   // Section of AOI that controls reading of the Status parameter (index 67).
   // ************************************************************************************************************
   40: XIO(Command_Being_Processed)XIO(Local_Control.4)EQU(Q90RKU.Command,12)OTL(Command_Being_Processed)MOV(Port,Port_Data.Data_Transfer[185])MOV(0,Port_Data.Data_Transfer[187])MOV(67,Port_Data.Data_Transfer[188])MOV(22,Port_Data.Data_Transfer[189])OTL(Port_Data.Port_Read.[Port])OTL(Local_Control.4);
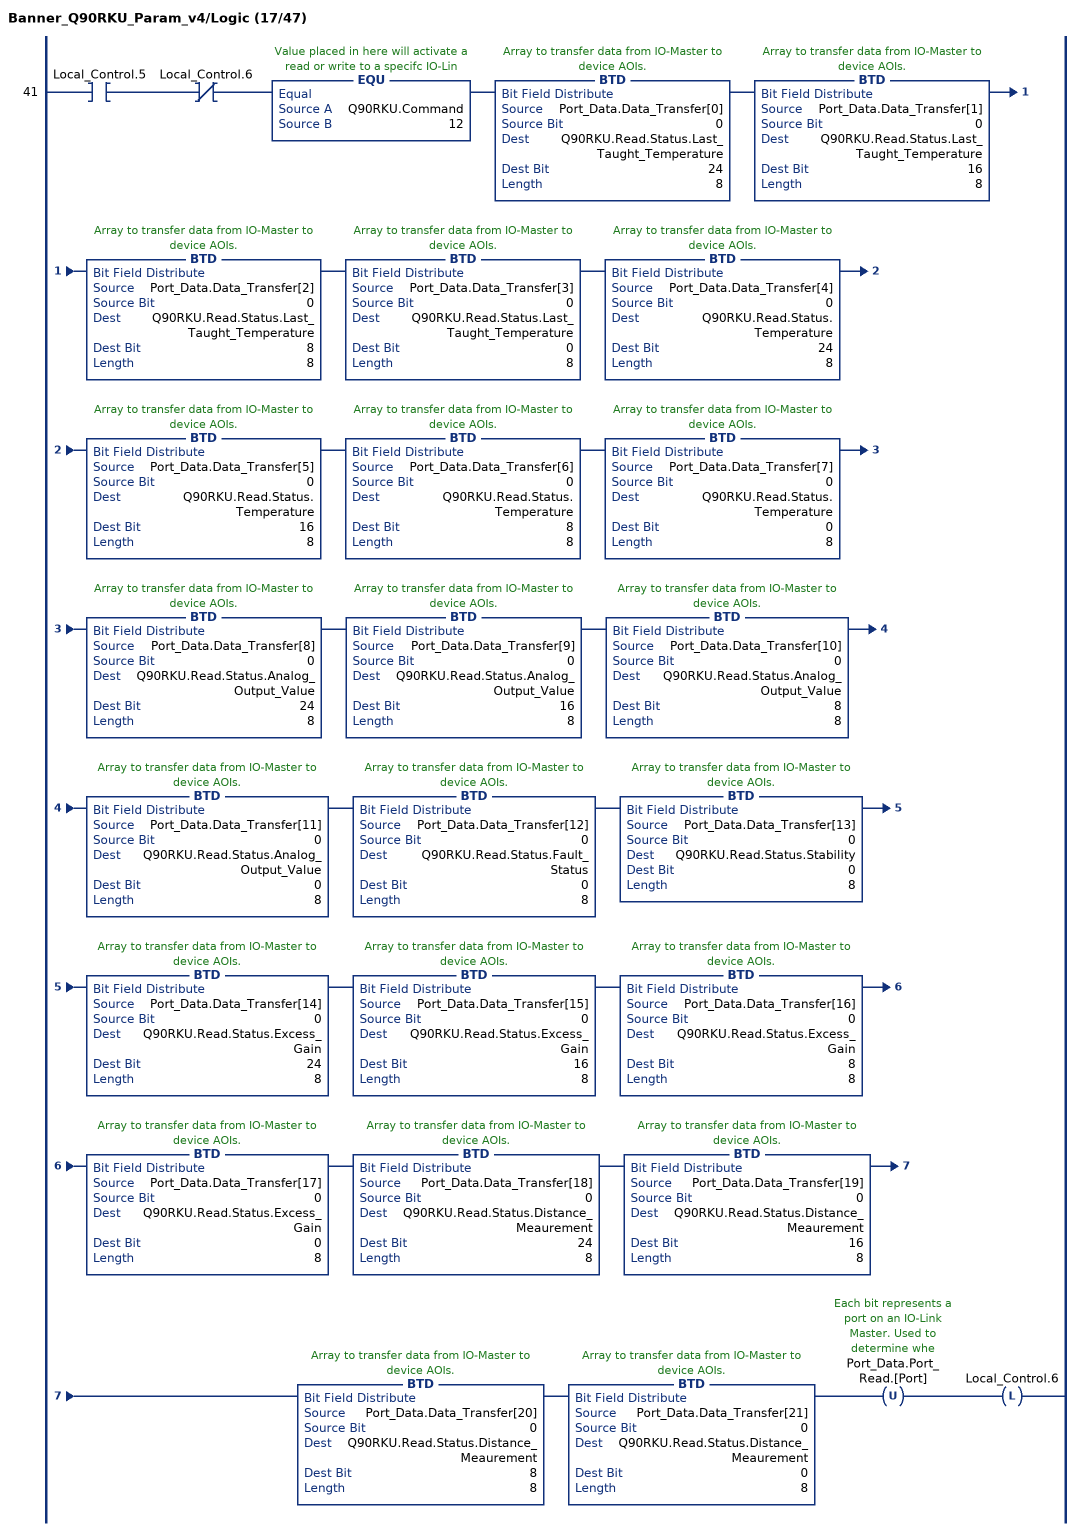
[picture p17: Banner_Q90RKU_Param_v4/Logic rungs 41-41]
   41: XIC(Local_Control.5)XIO(Local_Control.6)EQU(Q90RKU.Command,12)BTD(Port_Data.Data_Transfer[0],0,Q90RKU.Read.Status.Last_Taught_Temperature,24,8)BTD(Port_Data.Data_Transfer[1],0,Q90RKU.Read.Status.Last_Taught_Temperature,16,8)BTD(Port_Data.Data_Transfer[2],0,Q90RKU.Read.Status.Last_Taught_Temperature,8,8)BTD(Port_Data.Data_Transfer[3],0,Q90RKU.Read.Status.Last_Taught_Temperature,0,8)BTD(Port_Data.Data_Transfer[4],0,Q90RKU.Read.Status.Temperature,24,8)BTD(Port_Data.Data_Transfer[5],0,Q90RKU.Read.Status.Temperature,16,8)BTD(Port_Data.Data_Transfer[6],0,Q90RKU.Read.Status.Temperature,8,8)BTD(Port_Data.Data_Transfer[7],0,Q90RKU.Read.Status.Temperature,0,8)BTD(Port_Data.Data_Transfer[8],0,Q90RKU.Read.Status.Analog_Output_Value,24,8)BTD(Port_Data.Data_Transfer[9],0,Q90RKU.Read.Status.Analog_Output_Value,16,8)BTD(Port_Data.Data_Transfer[10],0,Q90RKU.Read.Status.Analog_Output_Value,8,8)BTD(Port_Data.Data_Transfer[11],0,Q90RKU.Read.Status.Analog_Output_Value,0,8)BTD(Port_Data.Data_Transfer[12],0,Q90RKU.Read.Status.Fault_Status,0,8)BTD(Port_Data.Data_Transfer[13],0,Q90RKU.Read.Status.Stability,0,8)BTD(Port_Data.Data_Transfer[14],0,Q90RKU.Read.Status.Excess_Gain,24,8)BTD(Port_Data.Data_Transfer[15],0,Q90RKU.Read.Status.Excess_Gain,16,8)BTD(Port_Data.Data_Transfer[16],0,Q90RKU.Read.Status.Excess_Gain,8,8)BTD(Port_Data.Data_Transfer[17],0,Q90RKU.Read.Status.Excess_Gain,0,8)BTD(Port_Data.Data_Transfer[18],0,Q90RKU.Read.Status.Distance_Meaurement,24,8)BTD(Port_Data.Data_Transfer[19],0,Q90RKU.Read.Status.Distance_Meaurement,16,8)BTD(Port_Data.Data_Transfer[20],0,Q90RKU.Read.Status.Distance_Meaurement,8,8)BTD(Port_Data.Data_Transfer[21],0,Q90RKU.Read.Status.Distance_Meaurement,0,8)OTU(Port_Data.Port_Read.[Port])OTL(Local_Control.6);
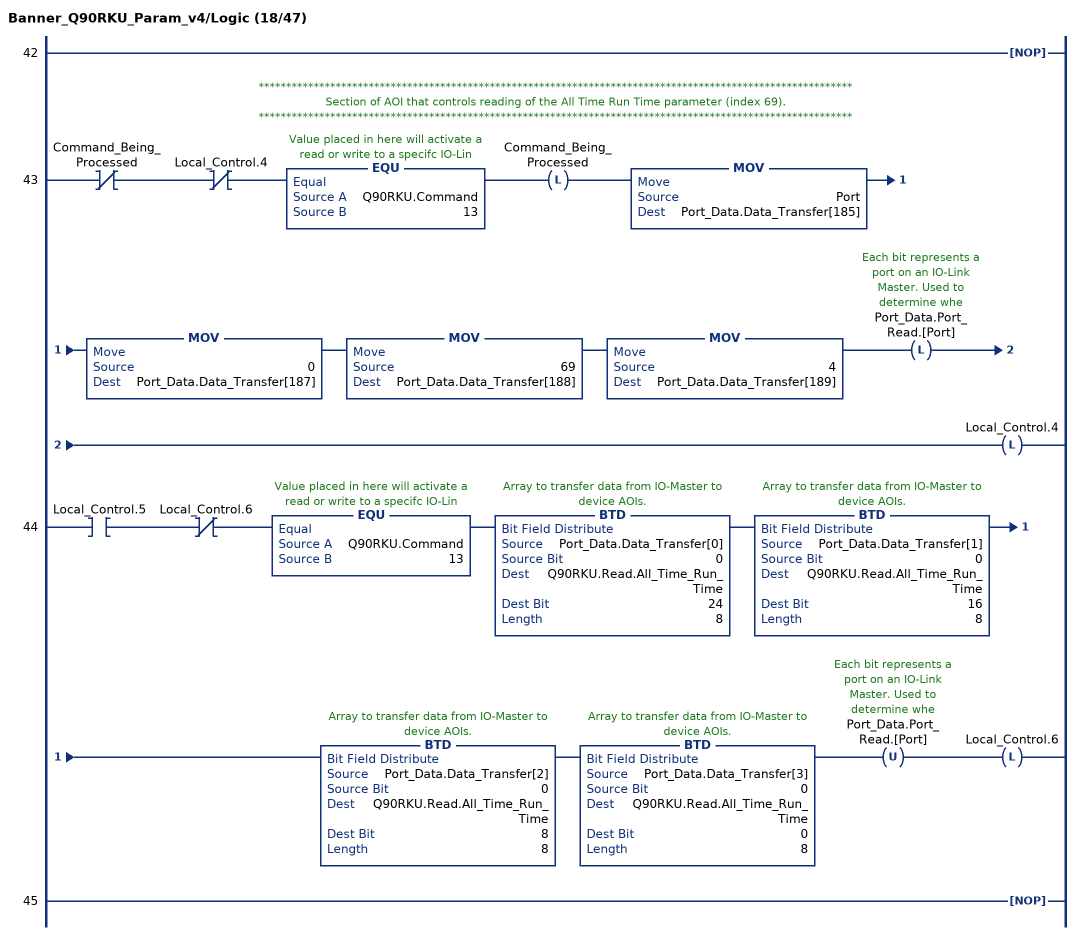
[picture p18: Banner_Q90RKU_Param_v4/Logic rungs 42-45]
   42: NOP();
   // ************************************************************************************************************
   // Section of AOI that controls reading of the All Time Run Time parameter (index 69).
   // ************************************************************************************************************
   43: XIO(Command_Being_Processed)XIO(Local_Control.4)EQU(Q90RKU.Command,13)OTL(Command_Being_Processed)MOV(Port,Port_Data.Data_Transfer[185])MOV(0,Port_Data.Data_Transfer[187])MOV(69,Port_Data.Data_Transfer[188])MOV(4,Port_Data.Data_Transfer[189])OTL(Port_Data.Port_Read.[Port])OTL(Local_Control.4);
   44: XIC(Local_Control.5)XIO(Local_Control.6)EQU(Q90RKU.Command,13)BTD(Port_Data.Data_Transfer[0],0,Q90RKU.Read.All_Time_Run_Time,24,8)BTD(Port_Data.Data_Transfer[1],0,Q90RKU.Read.All_Time_Run_Time,16,8)BTD(Port_Data.Data_Transfer[2],0,Q90RKU.Read.All_Time_Run_Time,8,8)BTD(Port_Data.Data_Transfer[3],0,Q90RKU.Read.All_Time_Run_Time,0,8)OTU(Port_Data.Port_Read.[Port])OTL(Local_Control.6);
   45: NOP();
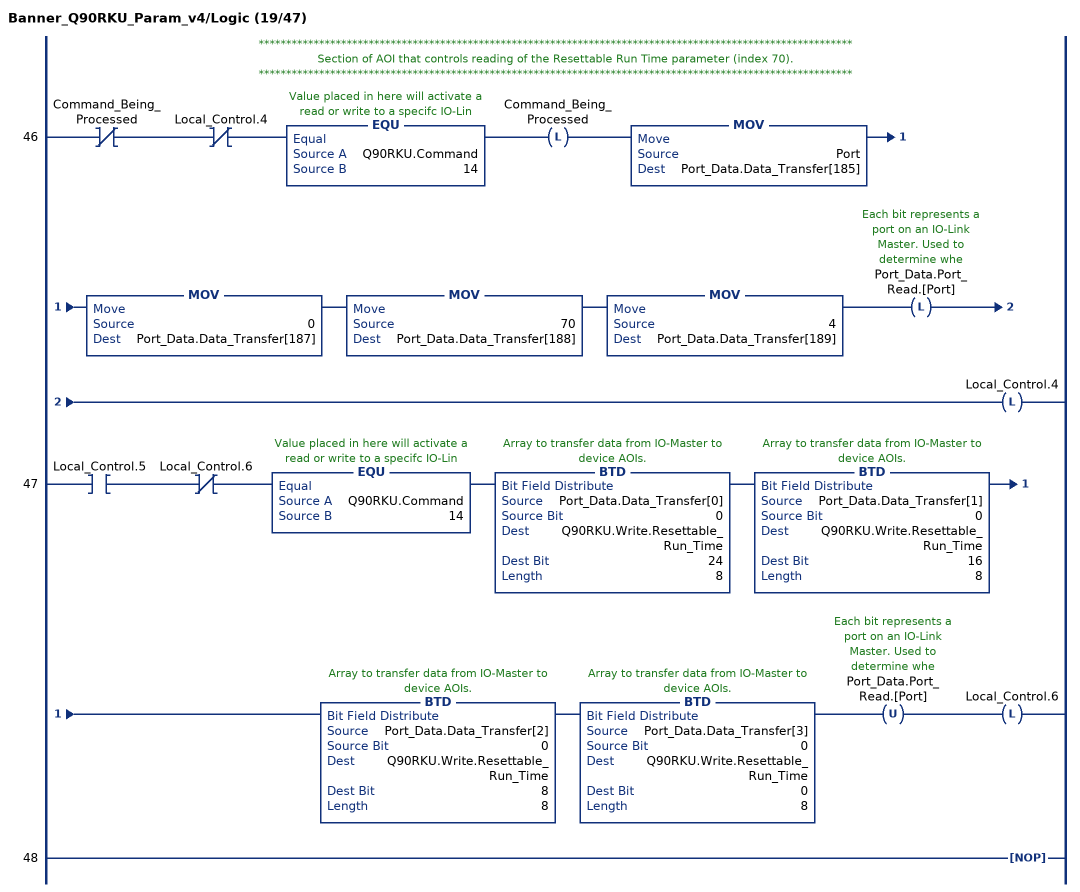
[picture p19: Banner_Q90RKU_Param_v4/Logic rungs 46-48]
   // ************************************************************************************************************
   // Section of AOI that controls reading of the Resettable Run Time parameter (index 70).
   // ************************************************************************************************************
   46: XIO(Command_Being_Processed)XIO(Local_Control.4)EQU(Q90RKU.Command,14)OTL(Command_Being_Processed)MOV(Port,Port_Data.Data_Transfer[185])MOV(0,Port_Data.Data_Transfer[187])MOV(70,Port_Data.Data_Transfer[188])MOV(4,Port_Data.Data_Transfer[189])OTL(Port_Data.Port_Read.[Port])OTL(Local_Control.4);
   47: XIC(Local_Control.5)XIO(Local_Control.6)EQU(Q90RKU.Command,14)BTD(Port_Data.Data_Transfer[0],0,Q90RKU.Write.Resettable_Run_Time,24,8)BTD(Port_Data.Data_Transfer[1],0,Q90RKU.Write.Resettable_Run_Time,16,8)BTD(Port_Data.Data_Transfer[2],0,Q90RKU.Write.Resettable_Run_Time,8,8)BTD(Port_Data.Data_Transfer[3],0,Q90RKU.Write.Resettable_Run_Time,0,8)OTU(Port_Data.Port_Read.[Port])OTL(Local_Control.6);
   48: NOP();
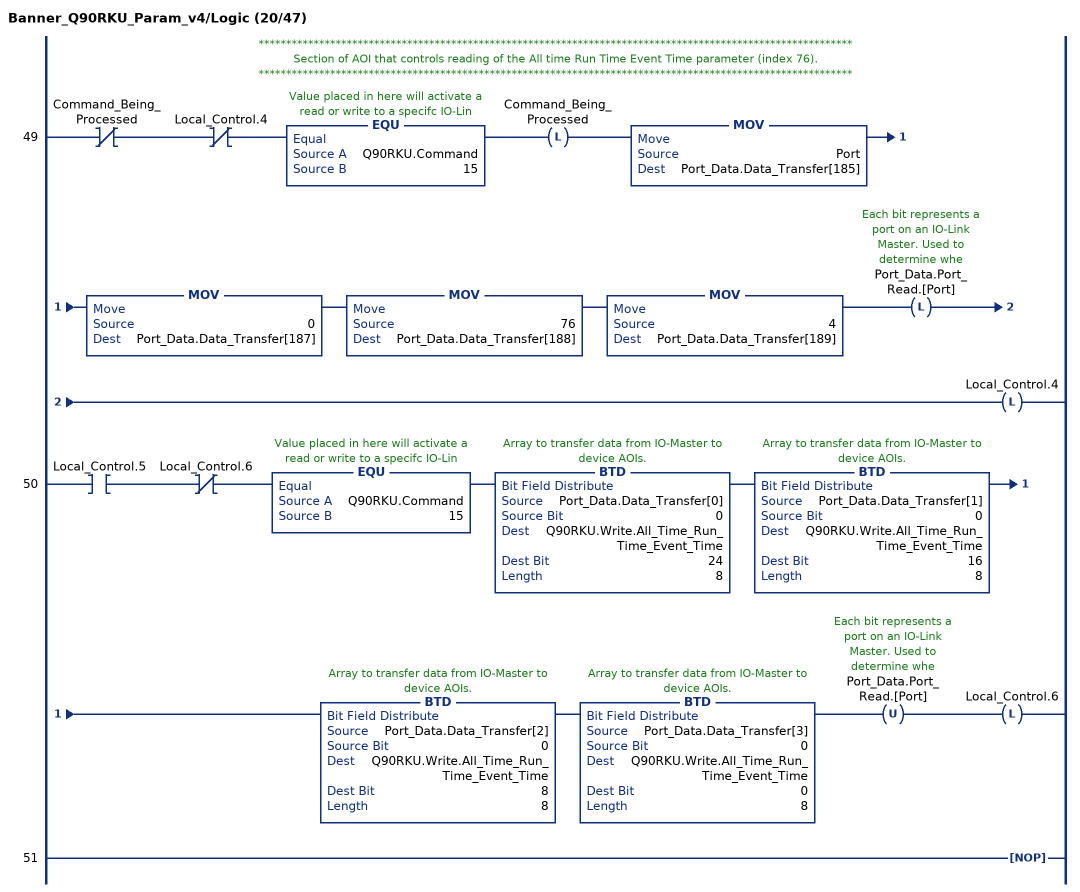
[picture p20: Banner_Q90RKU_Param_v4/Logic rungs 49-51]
   // ************************************************************************************************************
   // Section of AOI that controls reading of the All time Run Time Event Time parameter (index 76).
   // ************************************************************************************************************
   49: XIO(Command_Being_Processed)XIO(Local_Control.4)EQU(Q90RKU.Command,15)OTL(Command_Being_Processed)MOV(Port,Port_Data.Data_Transfer[185])MOV(0,Port_Data.Data_Transfer[187])MOV(76,Port_Data.Data_Transfer[188])MOV(4,Port_Data.Data_Transfer[189])OTL(Port_Data.Port_Read.[Port])OTL(Local_Control.4);
   50: XIC(Local_Control.5)XIO(Local_Control.6)EQU(Q90RKU.Command,15)BTD(Port_Data.Data_Transfer[0],0,Q90RKU.Write.All_Time_Run_Time_Event_Time,24,8)BTD(Port_Data.Data_Transfer[1],0,Q90RKU.Write.All_Time_Run_Time_Event_Time,16,8)BTD(Port_Data.Data_Transfer[2],0,Q90RKU.Write.All_Time_Run_Time_Event_Time,8,8)BTD(Port_Data.Data_Transfer[3],0,Q90RKU.Write.All_Time_Run_Time_Event_Time,0,8)OTU(Port_Data.Port_Read.[Port])OTL(Local_Control.6);
   51: NOP();
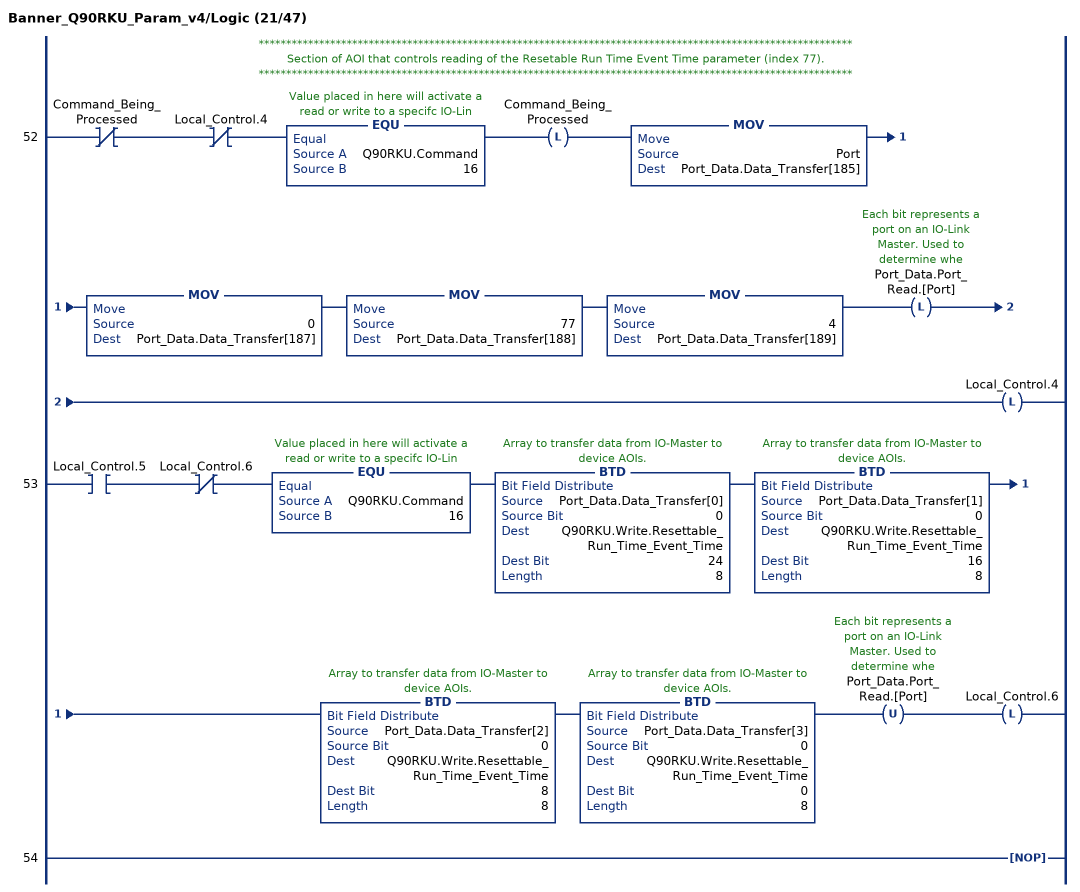
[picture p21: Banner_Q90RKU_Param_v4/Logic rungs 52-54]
   // ************************************************************************************************************
   // Section of AOI that controls reading of the Resetable Run Time Event Time parameter (index 77).
   // ************************************************************************************************************
   52: XIO(Command_Being_Processed)XIO(Local_Control.4)EQU(Q90RKU.Command,16)OTL(Command_Being_Processed)MOV(Port,Port_Data.Data_Transfer[185])MOV(0,Port_Data.Data_Transfer[187])MOV(77,Port_Data.Data_Transfer[188])MOV(4,Port_Data.Data_Transfer[189])OTL(Port_Data.Port_Read.[Port])OTL(Local_Control.4);
   53: XIC(Local_Control.5)XIO(Local_Control.6)EQU(Q90RKU.Command,16)BTD(Port_Data.Data_Transfer[0],0,Q90RKU.Write.Resettable_Run_Time_Event_Time,24,8)BTD(Port_Data.Data_Transfer[1],0,Q90RKU.Write.Resettable_Run_Time_Event_Time,16,8)BTD(Port_Data.Data_Transfer[2],0,Q90RKU.Write.Resettable_Run_Time_Event_Time,8,8)BTD(Port_Data.Data_Transfer[3],0,Q90RKU.Write.Resettable_Run_Time_Event_Time,0,8)OTU(Port_Data.Port_Read.[Port])OTL(Local_Control.6);
   54: NOP();
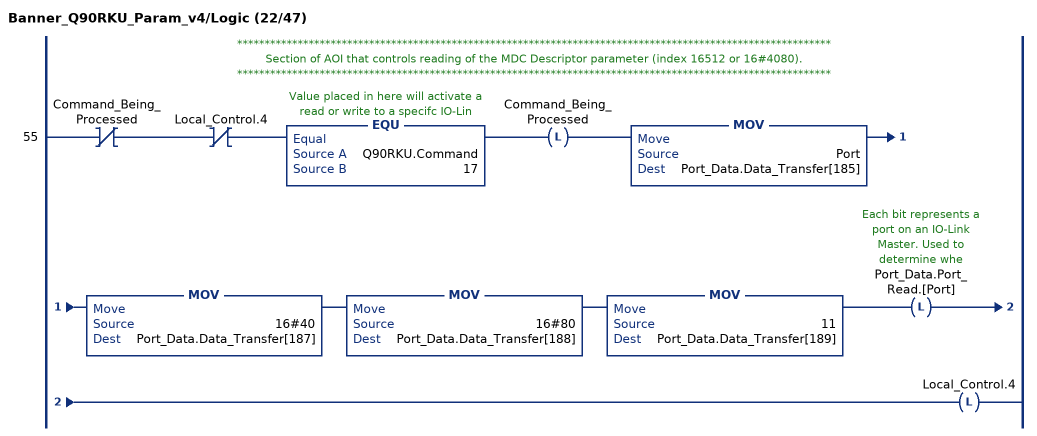
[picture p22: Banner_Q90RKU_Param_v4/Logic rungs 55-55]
   // ************************************************************************************************************
   // Section of AOI that controls reading of the MDC Descriptor parameter (index 16512 or 16#4080).
   // ************************************************************************************************************
   55: XIO(Command_Being_Processed)XIO(Local_Control.4)EQU(Q90RKU.Command,17)OTL(Command_Being_Processed)MOV(Port,Port_Data.Data_Transfer[185])MOV(16#40,Port_Data.Data_Transfer[187])MOV(16#80,Port_Data.Data_Transfer[188])MOV(11,Port_Data.Data_Transfer[189])OTL(Port_Data.Port_Read.[Port])OTL(Local_Control.4);
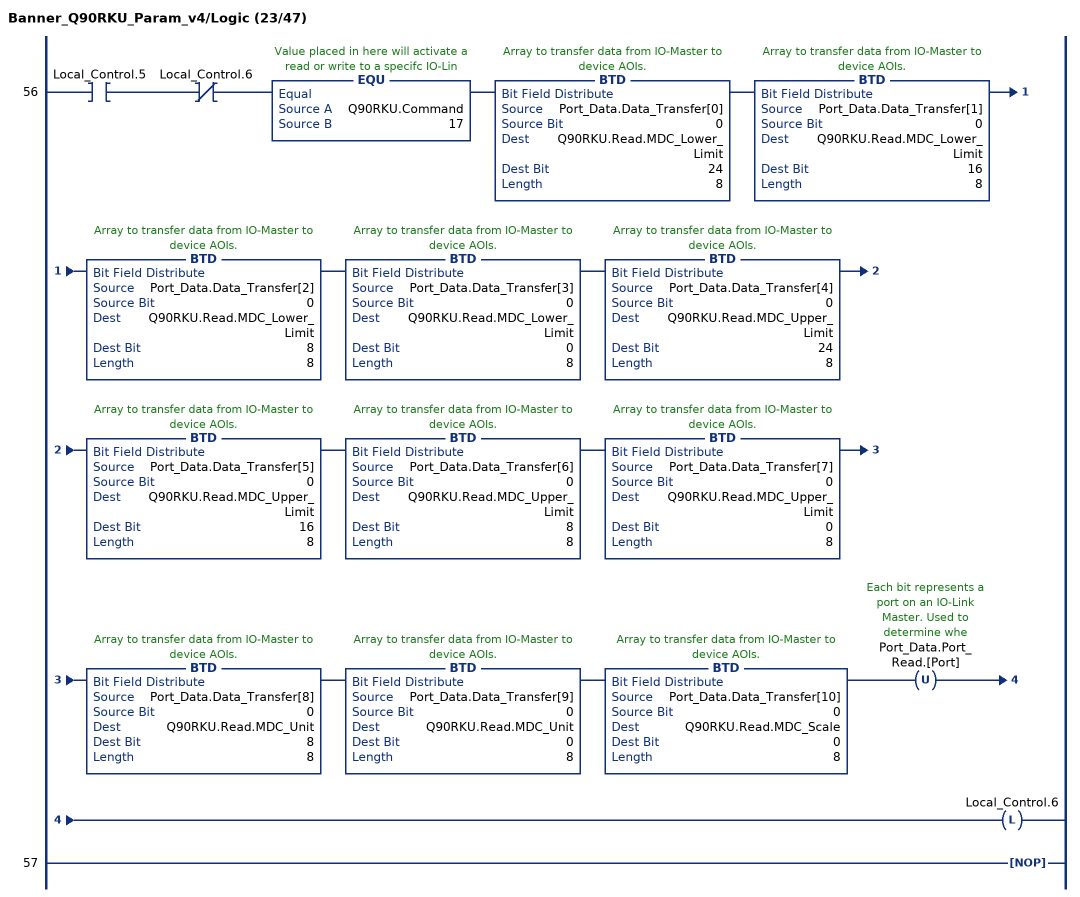
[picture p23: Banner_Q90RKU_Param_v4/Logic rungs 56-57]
   56: XIC(Local_Control.5)XIO(Local_Control.6)EQU(Q90RKU.Command,17)BTD(Port_Data.Data_Transfer[0],0,Q90RKU.Read.MDC_Lower_Limit,24,8)BTD(Port_Data.Data_Transfer[1],0,Q90RKU.Read.MDC_Lower_Limit,16,8)BTD(Port_Data.Data_Transfer[2],0,Q90RKU.Read.MDC_Lower_Limit,8,8)BTD(Port_Data.Data_Transfer[3],0,Q90RKU.Read.MDC_Lower_Limit,0,8)BTD(Port_Data.Data_Transfer[4],0,Q90RKU.Read.MDC_Upper_Limit,24,8)BTD(Port_Data.Data_Transfer[5],0,Q90RKU.Read.MDC_Upper_Limit,16,8)BTD(Port_Data.Data_Transfer[6],0,Q90RKU.Read.MDC_Upper_Limit,8,8)BTD(Port_Data.Data_Transfer[7],0,Q90RKU.Read.MDC_Upper_Limit,0,8)BTD(Port_Data.Data_Transfer[8],0,Q90RKU.Read.MDC_Unit,8,8)BTD(Port_Data.Data_Transfer[9],0,Q90RKU.Read.MDC_Unit,0,8)BTD(Port_Data.Data_Transfer[10],0,Q90RKU.Read.MDC_Scale,0,8)OTU(Port_Data.Port_Read.[Port])OTL(Local_Control.6);
   57: NOP();
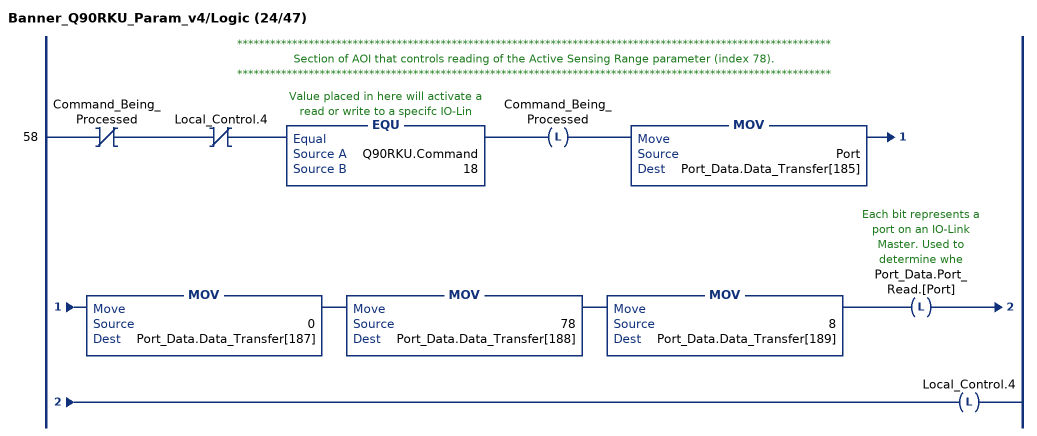
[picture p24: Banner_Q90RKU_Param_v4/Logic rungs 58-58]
   // ************************************************************************************************************
   // Section of AOI that controls reading of the Active Sensing Range parameter (index 78).
   // ************************************************************************************************************
   58: XIO(Command_Being_Processed)XIO(Local_Control.4)EQU(Q90RKU.Command,18)OTL(Command_Being_Processed)MOV(Port,Port_Data.Data_Transfer[185])MOV(0,Port_Data.Data_Transfer[187])MOV(78,Port_Data.Data_Transfer[188])MOV(8,Port_Data.Data_Transfer[189])OTL(Port_Data.Port_Read.[Port])OTL(Local_Control.4);
